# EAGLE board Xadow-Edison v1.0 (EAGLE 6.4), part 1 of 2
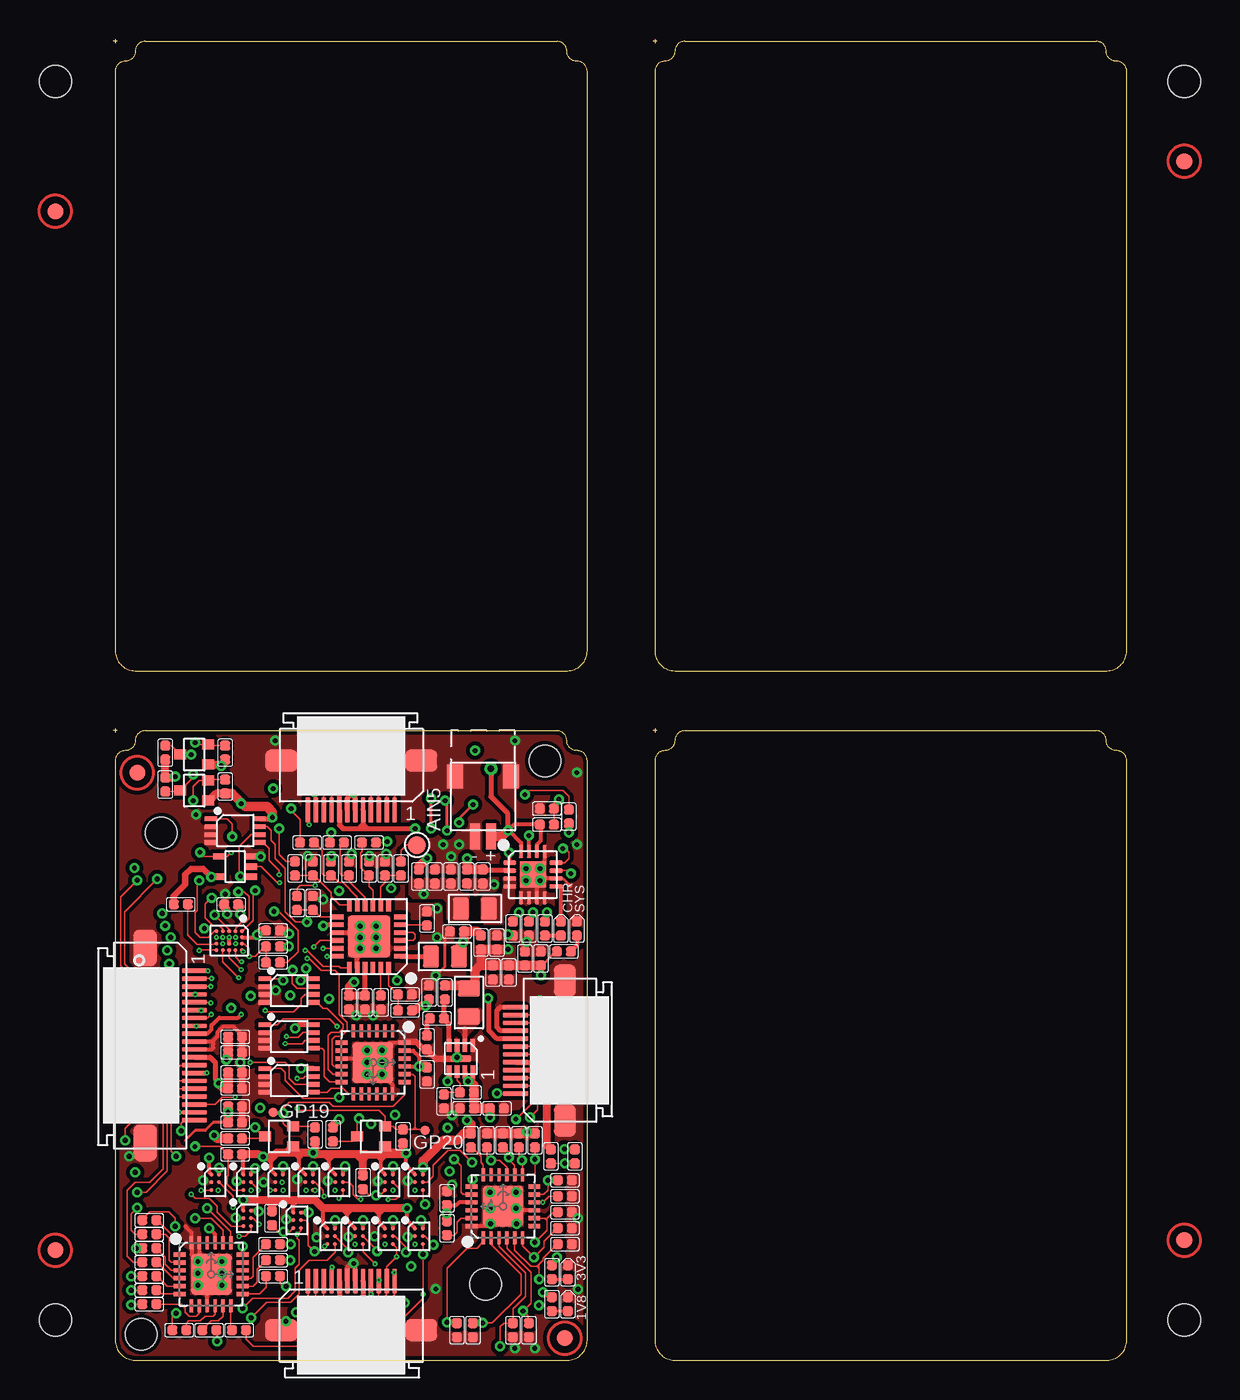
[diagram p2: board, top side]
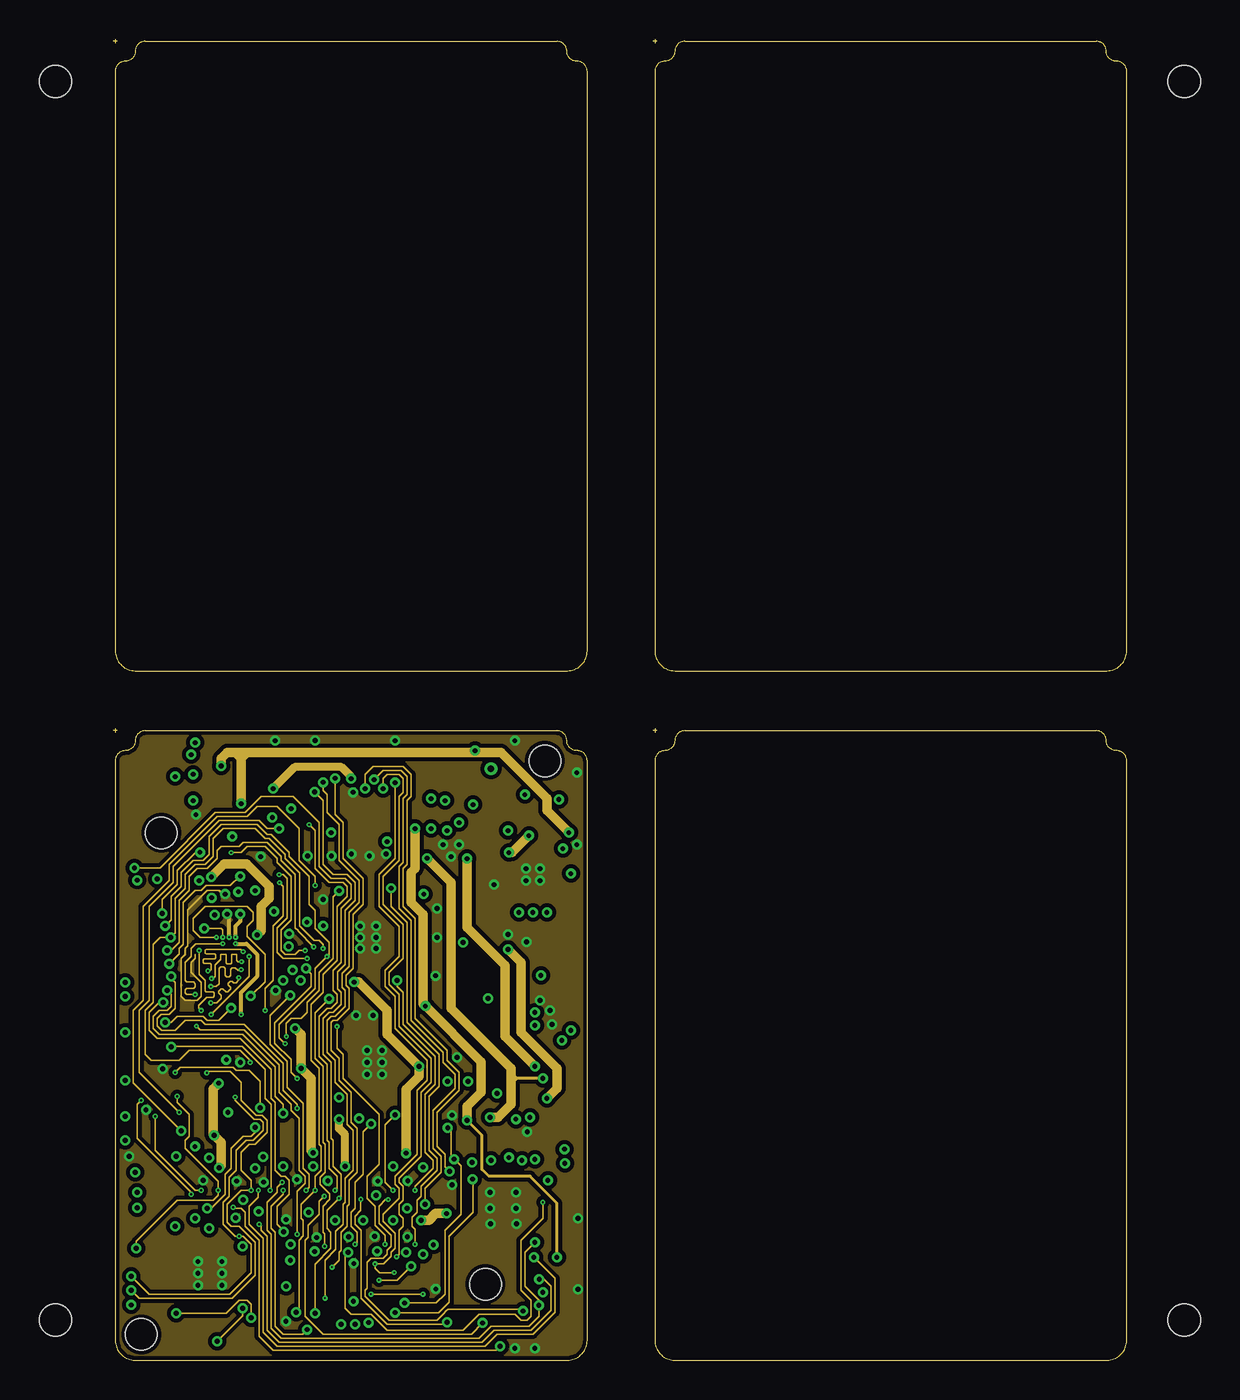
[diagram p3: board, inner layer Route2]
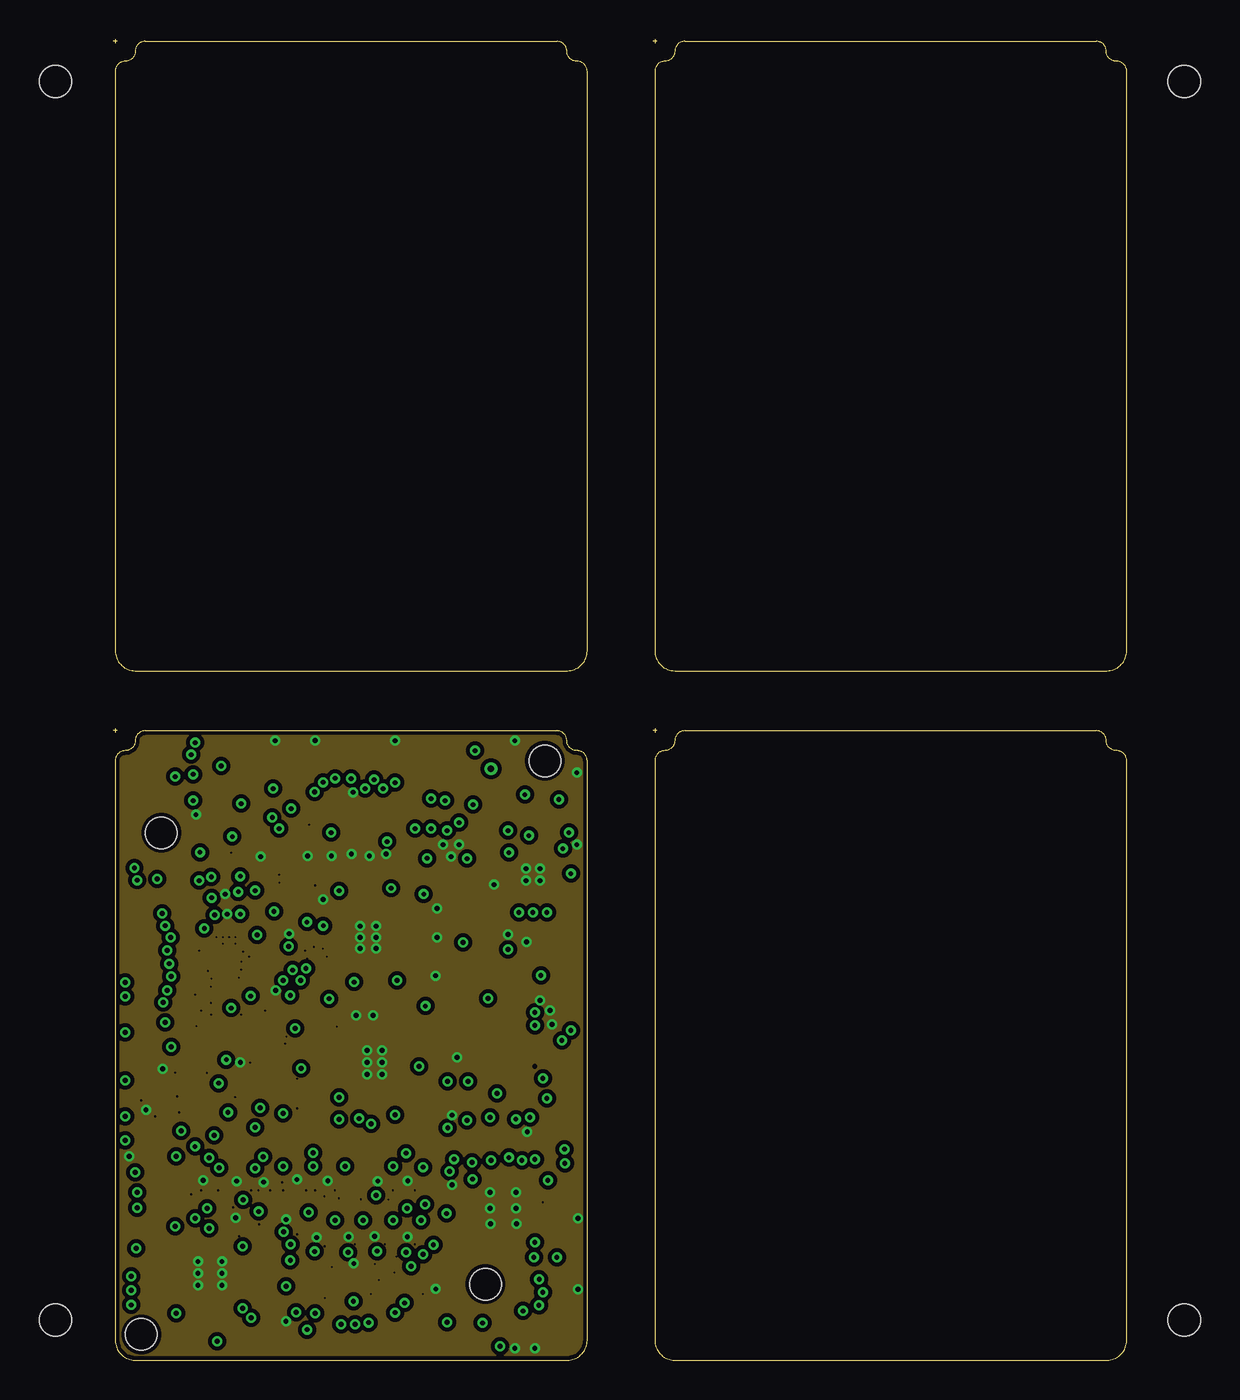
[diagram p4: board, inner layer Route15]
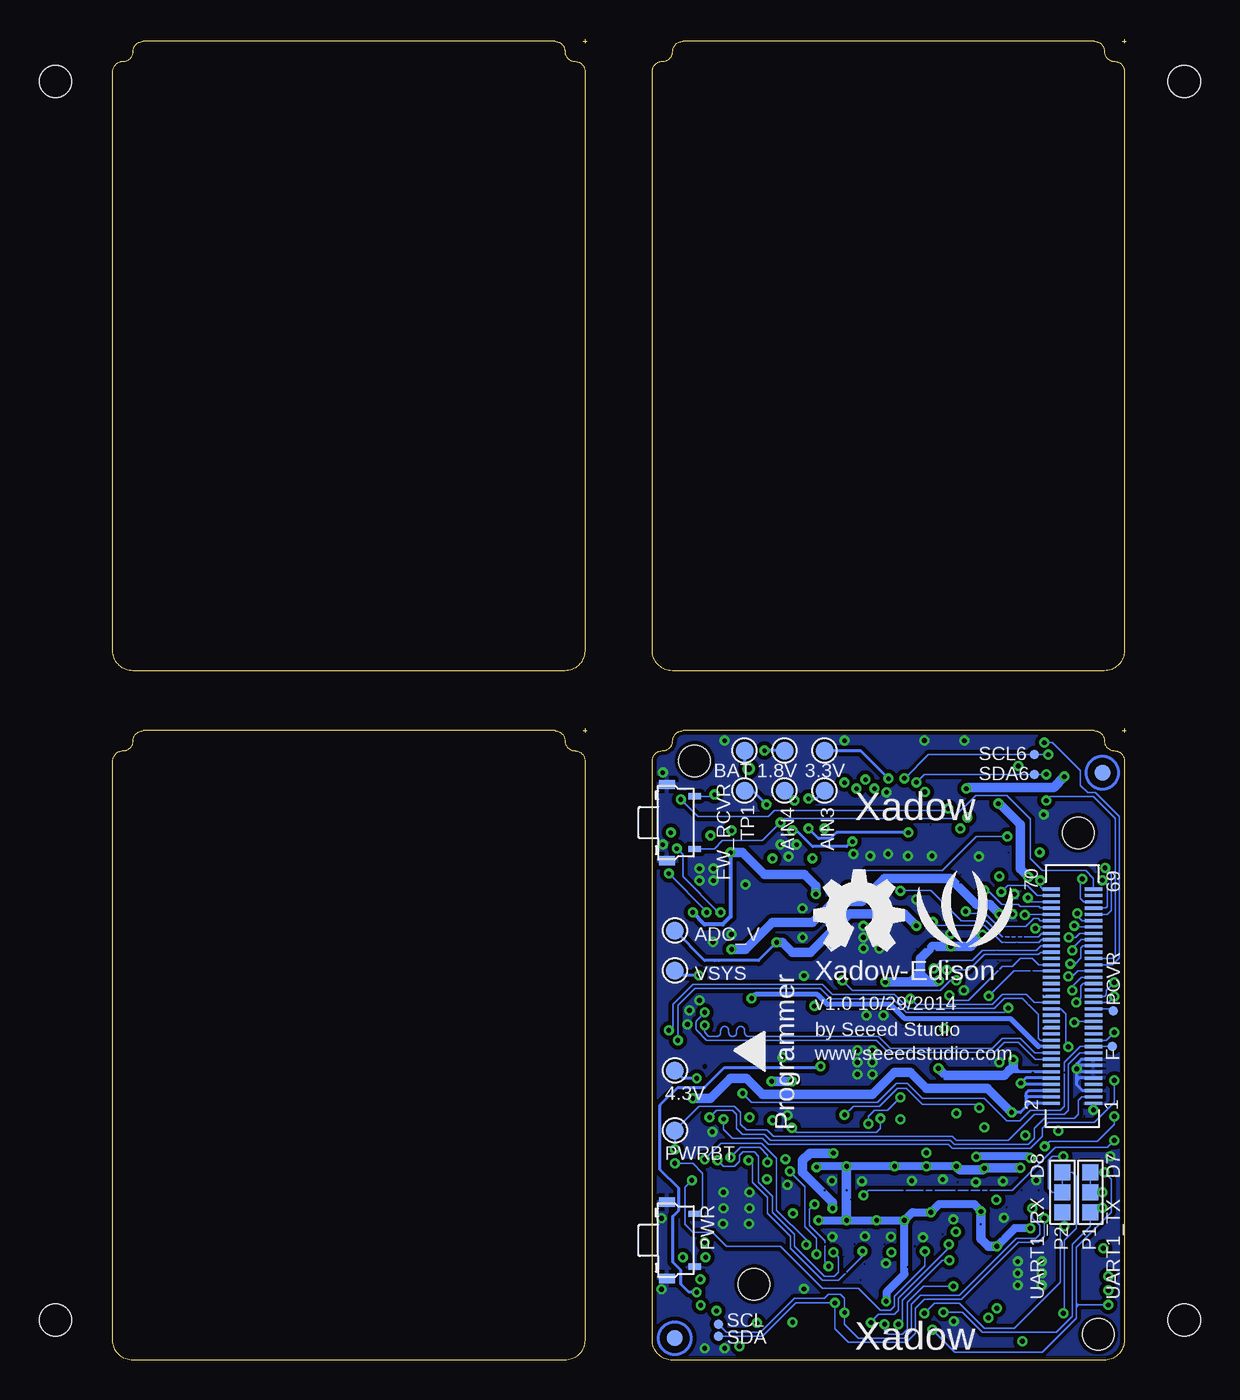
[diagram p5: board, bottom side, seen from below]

Size 64.42 x 83.95 mm. Coordinates in mm from the lower left corner, seen from the top.
Outline: 69 segments
Copper layers [2:(1+(2*15)+16):15]: Top 0.035mm / dielectric 0.2mm / Route2 0.0175mm / dielectric 0.3mm / Route15 0.0175mm / dielectric 0.2mm / Bottom 0.035mm
Design rules "SeeedStudio_4layer_DRU_no_angle_20140221 *": minimum track width 4mil, minimum drill 4mil, track to track 6mil, track to pad 6mil, pad to pad 6mil, via to via 6mil, smd to smd 0mil, copper to edge 10mil, drill to drill 10mil, minimum pad ring 6mil, minimum via ring 4mil, stop-mask expansion 2mil, vias tented up to drill 25mil, thermal gap 10mil
Holes 2 mm at 3.06,33.52 23.66,4.83 27.44,38.09 1.79,1.64
Holes 2.03 mm at -3.68,81.28 -3.68,2.54 68.07,81.28 68.07,2.54
tKeepout: area 21.8,2.9 to 25.6,6.7; area 1.2,31.6 to 5,35.4
bKeepout: area 1.2,31.6 to 5,35.4
tRestrict: area 22.9,28.1 to 23,29.2; area 22,22.7 to 23.2,22.8; area 21,25.1 to 21.1,26.2

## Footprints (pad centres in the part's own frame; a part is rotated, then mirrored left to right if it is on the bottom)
TP-D45MIL = smd 1.143 x 1.143: T 0,0
LED-0402 = smd 0.635 x 0.635: + -0.445,0; - 0.445,0
C0402 = smd 0.635 x 0.635: 1 -0.445,0; 2 0.445,0
TP-D23MIL = smd 0.6 x 0.6: T 0,0
4P-SMD-L4.5*W3.8*H1.8MM-90D = smd 0.4 x 0.8: 1 -1.675,-1.277; 2 1.675,-1.277 | smd 0.6 x 1: S1 -2.425,0.5; S2 2.425,0.5
70PIN-SMD-L16.64*W3.38*H3.12MM = smd 0.2 x 1.1: 1 -6.8,-1.34; 2 -6.8,1.34; 3 -6.4,-1.34; 4 -6.4,1.34; 5 -6,-1.34; 6 -6,1.34; 7 -5.6,-1.34; 8 -5.6,1.34; 9 -5.2,-1.34; 10 -5.2,1.34; 11 -4.8,-1.34; 12 -4.8,1.34; 13 -4.4,-1.34; 14 -4.4,1.34; 15 -4,-1.34; 16 -4,1.34; 17 -3.6,-1.34; 18 -3.6,1.34; 19 -3.2,-1.34; 20 -3.2,1.34; 21 -2.8,-1.34; 22 -2.8,1.34; 23 -2.4,-1.34; 24 -2.4,1.34; 25 -2,-1.34; 26 -2,1.34; 27 -1.6,-1.34; 28 -1.6,1.34; 29 -1.2,-1.34; 30 -1.2,1.34; 31 -0.8,-1.34; 32 -0.8,1.34; 33 -0.4,-1.34; 34 -0.4,1.34; 35 0,-1.34; 36 0,1.34; 37 0.4,-1.34; 38 0.4,1.34; 39 0.8,-1.34; 40 0.8,1.34; 41 1.2,-1.34; 42 1.2,1.34; 43 1.6,-1.34; 44 1.6,1.34; 45 2,-1.34; 46 2,1.34; 47 2.4,-1.34; 48 2.4,1.34; 49 2.8,-1.34; 50 2.8,1.34; 51 3.2,-1.34; 52 3.2,1.34; 53 3.6,-1.34; 54 3.6,1.34; 55 4,-1.34; 56 4,1.34; 57 4.4,-1.34; 58 4.4,1.34; 59 4.8,-1.34; 60 4.8,1.34; 61 5.2,-1.34; 62 5.2,1.34; 63 5.6,-1.34; 64 5.6,1.34; 65 6,-1.34; 66 6,1.34; 67 6.4,-1.34; 68 6.4,1.34; 69 6.8,-1.34; 70 6.8,1.34
20P-0.5 = smd 0.3 x 1.6: 1 -4.75,3.127; 2 -4.25,3.127; 3 -3.75,3.127; 4 -3.25,3.127; 5 -2.75,3.127; 6 -2.25,3.127; 7 -1.75,3.127; 8 -1.25,3.127; 9 -0.75,3.127; 10 -0.25,3.127; 11 0.25,3.127; 12 0.75,3.127; 13 1.25,3.127; 14 1.75,3.127; 15 2.25,3.127; 16 2.75,3.127; 17 3.25,3.127; 18 3.75,3.127; 19 4.25,3.127; 20 4.75,3.127 | smd 2.3 x 1.5: P1 -6.2,0; P2 6.2,0
12P-0.5-NEW = smd 0.3 x 1.6: 1 -2.75,3.127; 2 -2.25,3.127; 3 -1.75,3.127; 4 -1.25,3.127; 5 -0.75,3.127; 6 -0.25,3.127; 7 0.25,3.127; 8 0.75,3.127; 9 1.25,3.127; 10 1.75,3.127; 11 2.25,3.127; 12 2.75,3.127 | smd 2.032 x 1.397: P1 -4.445,0; P2 4.445,0
2P-SMD-1.0-90D = smd 1.524 x 1.016: 3 -3.429,1.778; 4 -3.429,-1.778 | smd 1.651 x 0.635: + 0.381,0.508; - 0.381,-0.508
L0805 = smd 1.016 x 1.397: 1 -0.889,0; 2 0.889,0
3P-SMD-4.1X1.5 = smd 1.016 x 1.016: 00 -1.27,0; 11 1.27,0; MM 0,0
ROUND-MARK-1.0 = smd 1.016 x 1.016: P$1 0,0
SOT-323 = smd 0.635 x 0.762: 1 -0.635,-0.889; 2 0.635,-0.889; 3 0,0.889
R0402 = smd 0.635 x 0.635: 1 -0.445,0; 2 0.445,0
S-PVQFN-N24 = smd 0.8 x 0.3: 1 -2,1.25; 2 -2,0.75; 3 -2,0.25; 4 -2,-0.25; 5 -2,-0.75; 6 -2,-1.25; 13 2,-1.25; 14 2,-0.75; 15 2,-0.25; 16 2,0.25; 17 2,0.75; 18 2,1.25 | smd 0.3 x 0.8: 7 -1.25,-2; 8 -0.75,-2; 9 -0.25,-2; 10 0.25,-2; 11 0.75,-2; 12 1.25,-2; 19 1.25,2; 20 0.75,2; 21 0.25,2; 22 -0.25,2; 23 -0.75,2; 24 -1.25,2 | smd 2.7 x 2.7: P$25 0,0
R-XBGA-N6 = smd 0.25 x 0.25: 1 -0.25,0.5; 2 -0.25,0; 3 -0.25,-0.5; 4 0.25,-0.5; 5 0.25,0; 6 0.25,0.5
QFN24 = smd 0.8 x 0.26: 1 -2,1.25; 2 -2,0.75; 3 -2,0.25; 4 -2,-0.25; 5 -2,-0.75; 6 -2,-1.25; 13 2,-1.25; 14 2,-0.75; 15 2,-0.25; 16 2,0.25; 17 2,0.75; 18 2,1.25 | smd 0.26 x 0.8: 7 -1.25,-2; 8 -0.75,-2; 9 -0.25,-2; 10 0.25,-2; 11 0.75,-2; 12 1.25,-2; 19 1.25,2; 20 0.75,2; 21 0.25,2; 22 -0.25,2; 23 -0.75,2; 24 -1.25,2 | smd 2.6 x 2.6: E 0.02,-0.01
R-XBGA-N20 = smd 0.25 x 0.25: 1 -0.6,0.8; 2 -0.2,0.8; 3 0.2,0.8; 4 0.6,0.8; 5 -0.6,0.4; 6 -0.2,0.4; 7 0.2,0.4; 8 0.6,0.4; 9 -0.6,0; 10 -0.2,0; 11 0.2,0; 12 0.6,0; 13 -0.6,-0.4; 14 -0.2,-0.4; 15 0.2,-0.4; 16 0.6,-0.4; 17 -0.6,-0.8; 18 -0.2,-0.8; 19 0.2,-0.8; 20 0.6,-0.8
US-8 = smd 0.3 x 0.8: 1 -0.75,-1.55; 2 -0.25,-1.55; 3 0.25,-1.55; 4 0.75,-1.55; 5 0.75,1.55; 6 0.25,1.55; 7 -0.25,1.55; 8 -0.75,1.55
SOT-353 = smd 0.4 x 0.8: 1 -0.65,-1; 2 0,-1; 3 0.65,-1; 4 0.65,1; 5 -0.65,1
QFN16 = smd 0.85 x 0.28: 1 -1.475,0.75; 2 -1.475,0.25; 3 -1.475,-0.25; 4 -1.475,-0.75; 9 1.475,-0.75; 10 1.475,-0.25; 11 1.475,0.25; 12 1.475,0.75 | smd 0.28 x 0.85: 5 -0.75,-1.475; 6 -0.25,-1.475; 7 0.25,-1.475; 8 0.75,-1.475; 13 0.75,1.475; 14 0.25,1.475; 15 -0.25,1.475; 16 -0.75,1.475 | smd 1.65 x 1.65: PAD 0,0
DFN-8L = smd 0.8 x 0.3: 1 -0.827,0.75; 2 -0.827,0.25; 3 -0.827,-0.25; 4 -0.827,-0.75; 5 0.827,-0.75; 6 0.827,-0.25; 7 0.827,0.25; 8 0.827,0.75 | smd 0.45 x 1.3: 9 0,0

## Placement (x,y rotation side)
1.8V  [TP-D45MIL]  21.72,38.73 0 bottom
1V8  red  [LED-0402]  28.89,3.56 90 top
3.3V  [TP-D45MIL]  19.18,38.73 0 bottom
3V3  blue  [LED-0402]  28.89,5.59 90 top
4.3V  [TP-D45MIL]  28.7,18.41 0 bottom
ADC_V  [TP-D45MIL]  28.7,27.3 0 bottom
AIN3  [TP-D45MIL]  19.18,36.2 0 bottom
AIN4  [TP-D45MIL]  21.72,36.2 0 bottom
AIN5  [TP-D45MIL]  19.3,32.74 0 top
BAT  [TP-D45MIL]  24.26,38.73 0 bottom
C3  10uF  [C0402]  14.99,22.73 270 top
C4  100nF  [C0402]  16,22.73 270 top
C5  10uF  [C0402]  21.84,27.24 180 top
C6  100nF  [C0402]  24.38,26.54 90 top
C7  10uF  [C0402]  20.07,23.37 90 top
C8  100pF  [C0402]  12.7,29.06 270 top
C9  100pF  [C0402]  12.7,31.24 270 top
C10  100pF  [C0402]  13.84,31.24 270 top
C11  100pF  [C0402]  14.99,31.24 270 top
C12  100pF  [C0402]  16.26,31.24 270 top
C13  100pF  [C0402]  17.27,31.24 270 top
C14  100nF  [C0402]  10.16,27.3 0 top
C15  100nF  [C0402]  7.49,28.96 180 top
C16  100nF  [C0402]  21.21,10.29 90 top
C17  100nF  [C0402]  19.94,18.16 270 top
C19  10uF  [C0402]  25.15,24.64 270 top
C20  10uF  [C0402]  24.13,24.64 270 top
C21  100nF  [C0402]  26.16,25.53 90 top
C22  100nF  [C0402]  27.18,25.53 90 top
C23  10uF  [C0402]  22.48,16 180 top
C24  10uF  [C0402]  24.38,16 0 top
C25  10uF  [C0402]  22.48,30.73 90 top
C26  10uF  [C0402]  23.49,30.73 90 top
C27  10uF  [C0402]  21.46,30.73 90 top
C28  10uF  [C0402]  20.45,30.73 90 top
C29  10uF  [C0402]  7.75,15.11 0 top
C30  10uF  [C0402]  7.75,16.13 0 top
C31  10uF  [C0402]  7.75,17.27 0 top
C32  10uF  [C0402]  7.75,18.29 0 top
C33  10uF  [C0402]  7.75,19.56 0 top
C34  10uF  [C0402]  7.75,20.55 0 top
CHR  green  [LED-0402]  28.45,27.43 90 top
F  [TP-D23MIL]  0.89,19.94 0 bottom
FW_RCVR  311020035  [4P-SMD-L4.5*W3.8*H1.8MM-90D]  28.7,34.16 90 bottom
GP19  [TP-D23MIL]  10.16,15.75 0 top
GP20  [TP-D23MIL]  19.81,14.61 0 top
J1  DF40C(2.0)-70DS-0.4V(51)  [70PIN-SMD-L16.64*W3.38*H3.12MM]  3.43,23.13 90 bottom
J2  FH12-20S-0.5SH(55)  [20P-0.5]  2.03,20 270 top
J3  320060003／／FH12-12S-0.5SH(55)  [12P-0.5-NEW]  15.13,1.91 0 top
J4  320060003／／FH12-12S-0.5SH(55)  [12P-0.5-NEW]  15.13,38.1 180 top
J8  320110054  [2P-SMD-1.0-90D]  23.49,33.66 270 top
J9  320060003／／FH12-12S-0.5SH(55)  [12P-0.5-NEW]  28.7,19.68 90 top
L1  120R  [L0805]  21.08,25.65 180 top
L2  2.2uH  [L0805]  22.61,22.73 90 top
L3  2.2uH  [L0805]  22.99,28.7 180 top
P1  [3P-SMD-4.1X1.5]  2.29,10.67 90 bottom
P2  [3P-SMD-4.1X1.5]  4.06,10.67 90 bottom
P3  DNP  [ROUND-MARK-1.0]  28.7,1.4 0 bottom
P4  [ROUND-MARK-1.0]  not placed on the board
P5  [ROUND-MARK-1.0]  not placed on the board
P6  [ROUND-MARK-1.0]  not placed on the board
P7  [ROUND-MARK-1.0]  not placed on the board
P11  DNP  [ROUND-MARK-1.0]  28.7,1.4 0 top
P12  √  [ROUND-MARK-1.0]  1.52,37.34 0 bottom
P13  √  [ROUND-MARK-1.0]  1.52,37.34 0 top
PCVR  [TP-D23MIL]  0.83,22.19 0 bottom
PWR  311020035  [4P-SMD-L4.5*W3.8*H1.8MM-90D]  28.7,7.62 90 bottom
PWRBT  [TP-D45MIL]  28.7,14.61 0 bottom
Q1  BSS138LT3G  [SOT-323]  16.38,14.22 90 top
Q2  BSS138LT3G  [SOT-323]  10.54,14.22 90 top
Q3  BSS138LT3G  [SOT-323]  5.14,36.2 90 top
Q4  BSS138LT3G  [SOT-323]  5.14,38.48 90 top
R1  47K_1%  [R0402]  20.57,21.72 180 top
R2  1.8K  [R0402]  7.11,36.45 270 top
R3  3.3K  [R0402]  3.3,36.58 90 top
R4  0R  [R0402]  19.94,28.07 90 top
R5  0R  [R0402]  17.02,22.73 270 top
R6  22K_1%  [R0402]  18.54,23.24 0 top
R7  22K_1%  [R0402]  18.54,22.23 0 top
R8  33R  [R0402]  11.68,29.06 90 top
R9  33R  [R0402]  11.56,31.24 90 top
R10  33R  [R0402]  12.32,32.89 180 top
R11  33R  [R0402]  14.22,32.89 180 top
R12  33R  [R0402]  16.26,32.89 0 top
R13  33R  [R0402]  18.29,31.24 90 top
R14  10K  [R0402]  4.29,28.97 180 top
R15  10K  [R0402]  10.16,26.29 180 top
R16  10K  [R0402]  21.84,1.91 90 top
R17  10K  [R0402]  22.86,1.91 90 top
R18  10K  [R0402]  28.7,10.41 0 top
R19  10K  [R0402]  26.8,13.97 90 top
R20  10K  [R0402]  25.78,13.97 90 top
R21  10K  [R0402]  24.77,13.97 90 top
R22  10K  [R0402]  23.75,13.97 90 top
R23  0R  [R0402]  10.16,25.27 0 top
R24  10K  [R0402]  22.48,17.02 180 top
R25  NC  [R0402]  21.02,16.45 270 top
R26  510K  [R0402]  21.08,23.37 270 top
R27  47K_1%  [R0402]  19.94,20.19 270 top
R28  5.1K  [R0402]  25.4,27.43 270 top
R29  5.1K  [R0402]  26.42,27.43 270 top
R30  47K  [R0402]  10.08,9.02 90 top
R31  470  [R0402]  27.43,27.43 270 top
R32  10K  [R0402]  27.81,12.95 270 top
R33  0R  [R0402]  19.43,30.73 270 top
R34  100R  [R0402]  29.34,12.95 90 top
R35  100R  [R0402]  28.96,34.54 270 top
R36  1.8K  [R0402]  7.11,38.61 270 top
R37  0R  [R0402]  23.37,26.54 90 top
R38  1.8K  [R0402]  27.88,5.59 270 top
R39  510R  [R0402]  27.88,3.56 270 top
R40  1.8K  [R0402]  18.41,14.22 270 top
R41  3.3K  [R0402]  13.97,14.35 90 top
R42  1.8K  [R0402]  12.83,14.35 270 top
R43  3.3K  [R0402]  7.75,14.1 180 top
R44  10K  [R0402]  21.21,8.38 90 top
R45  10K  [R0402]  22.73,13.97 90 top
R46  47K  [R0402]  15.88,11.3 90 top
R47  47K  [R0402]  7.75,13.08 0 top
R48  10K  [R0402]  28.7,7.37 180 top
R49  10K  [R0402]  28.7,9.4 180 top
R50  10K  [R0402]  28.7,8.38 180 top
R51  10K  [R0402]  26.42,1.91 90 top
R52  10K  [R0402]  28.7,11.43 0 top
R53  10K  [R0402]  25.4,1.91 90 top
R54  47K  [R0402]  10.16,7.37 0 top
R55  47K  [R0402]  10.16,6.35 0 top
R56  47K  [R0402]  10.16,5.33 0 top
R57  47K  [R0402]  8,1.91 0 top
R58  47K  [R0402]  4.19,1.91 180 top
R59  47K  [R0402]  2.29,8.89 0 top
R60  47K  [R0402]  2.29,8 0 top
R61  47K  [R0402]  2.29,3.56 0 top
R62  47K  [R0402]  2.29,5.33 0 top
R63  47K  [R0402]  2.29,7.11 0 top
R64  47K  [R0402]  6.1,1.91 0 top
R65  47K  [R0402]  2.29,6.22 0 top
R66  47K  [R0402]  2.29,4.45 0 top
R67  3.3K  [R0402]  3.3,38.61 270 top
R68  1M_1%  [R0402]  27.56,34.04 0 top
R69  1M_1%  [R0402]  27.56,35.05 180 top
R70  3.3K  [R0402]  28.64,25.97 0 top
SCL  [TP-D23MIL]  25.91,2.29 0 bottom
SCL6  [TP-D23MIL]  5.84,38.48 0 bottom
SDA  [TP-D23MIL]  25.91,1.52 0 bottom
SDA6  [TP-D23MIL]  5.84,37.21 0 bottom
SYS  White  [LED-0402]  29.46,27.43 90 top
TP1  [TP-D45MIL]  24.26,36.2 0 bottom
U2  ADS7951SBRGE  [S-PVQFN-N24]  16.26,26.92 180 top
U3  SN74LVC1T45YZPR  [R-XBGA-N6]  17.53,7.87 0 top
U4  PCAL9555AHF  [QFN24]  24.77,9.78 90 top
U5  SN74LVC1T45YZPR  [R-XBGA-N6]  19.43,11.3 0 top
U6  SN74LVC1T45YZPR  [R-XBGA-N6]  19.43,7.87 0 top
U7  SN74LVC1T45YZPR  [R-XBGA-N6]  11.68,8.89 0 top
U8  SN74LVC1T45YZPR  [R-XBGA-N6]  12.45,11.3 0 top
U9  SN74LVC1T45YZPR  [R-XBGA-N6]  14.35,11.3 0 top
U10  TXS0206-29YFPRB  [R-XBGA-N20]  7.37,26.67 270 top
U11  SN74LVC1T45YZPR  [R-XBGA-N6]  15.62,7.87 0 top
U12  SN74LVC2G53  [US-8]  11.18,17.78 270 top
U13  SN74AUP1G125DCKR  [SOT-353]  7.75,31.37 90 top
U14  SN74LVC2G53  [US-8]  11.18,20.57 270 top
U15  SN74LVC2G53  [US-8]  11.18,23.5 270 top
U16  SN74LVC2G53  [US-8]  7.75,33.66 270 top
U17  PCAL9555AHF  [QFN24]  16.51,18.92 270 top
U18  PCAL9535AHF  [QFN24]  6.22,5.46 0 top
U19  ETA6003Q3Q  [QFN16]  26.67,30.86 0 top
U22  SN74LVC1T45YZPR  [R-XBGA-N6]  17.53,11.3 0 top
U23  SN74LVC1T45YZPR  [R-XBGA-N6]  8.51,11.3 0 top
U24  SN74LVC1T45YZPR  [R-XBGA-N6]  10.54,11.3 0 top
U25  SN74LVC1T45YZPR  [R-XBGA-N6]  13.84,7.87 0 top
U26  SN74LVC1T45YZPR  [R-XBGA-N6]  6.48,11.3 0 top
U27  SN74LVC1T45YZPR  [R-XBGA-N6]  8.51,9.02 0 top
U28  ETA3410D2I-T  [DFN-8L]  22.1,19.18 270 top
U$13  [OSHW_FILLX200_NOTEXT]  19.81,26.04 0 bottom
U$14  [LOGO_SILK]  10.29,27.94 0 bottom
VSYS  [TP-D45MIL]  28.7,24.77 0 bottom

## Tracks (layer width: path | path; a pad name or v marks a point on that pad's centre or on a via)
ADC_VCC  (via drill 0.3 pad 0.64)
  Top 0.305: U2.14 13.41,27.67 v13.35,27.61
  Top 0.508: L1.1 21.97,26.29 v22.22,26.54
  Top 0.61: v22.22,26.54 22.29,26.61 C5.1 23.11,27.24 R37.2
  Bottom 0.203: v22.22,26.54 23.37,25.4 25.91,25.4 26.16,25.4 26.8,25.4 ADC_V.T
  Bottom 0.61: v22.22,26.54 21.84,26.54 21.21,25.91 20.07,25.91 17.6,28.37 14.11,28.37 v13.35,27.61
AIN0  (via drill 0.1 pad 0.25 layers 1-2, 0.3 pad 0.64)
  Top 0.102: R8.2 11.68,29.97 11.89,30.18 v12.83,30.18 | 4.57,15.24 4.52,15.24 4.32,15.04 v4.32,14.58
  Top 0.203: 4.57,15.24 J2.20
  Route2 0.102: v12.83,30.18 12.83,30.73 11.81,31.75 11.81,33.78 10.41,35.19 9.15,35.19 8.51,34.54 6.6,34.54 3.56,31.5 3.56,30.48 1.91,28.83 1.91,22.86 1.27,22.23 1.27,17.63 v4.32,14.58
AIN1  (via drill 0.1 pad 0.25 layers 1-2, 0.3 pad 0.64)
  Top 0.102: J2.19 v4.19,15.75 | R9.2 10.99,31.69 10.54,32.13 v10.54,33.78
  Route2 0.102: v10.54,33.78 9.78,33.78 9.27,34.29 6.73,34.29 3.81,31.37 3.81,30.35 2.29,28.83 2.29,22.86 1.65,22.23 1.65,18.29 v4.19,15.75
AIN2/BAT  (via drill 0.3 pad 0.64)
  Top 0.102: R68.2 R69.1 28,35.5 28.14,35.64 v28.32,35.64 | R10.2 11.88,34.35 11.3,34.92 v11.3,35.05
  Bottom 0.102: v11.3,35.05 11.43,34.92 22.35,34.92 22.73,34.54 27.23,34.54 v28.32,35.64
  pour Top (isolate 0.254, no thermals): 24.13,33.53 23.88,33.66 24,33.53
AIN3  (via drill 0.3 pad 0.64)
  Top 0.102: R11.2 13.78,33.47 v13.84,33.53
  Top 0.203: v20.19,33.78 v20.19,35.69
  Bottom 0.203: v13.84,33.53 18.41,33.53 18.8,33.15 19.56,33.15 v20.19,33.78 | v20.19,35.69 19.68,35.69 AIN3.T
AIN4  (via drill 0.3 pad 0.64)
  Top 0.102: R12.2 17.34,32.89 v17.4,32.96
  Top 0.203: v21.21,33.66 21.21,35.43 v21.08,35.56
  Bottom 0.203: AIN4.T v21.08,35.56 | v17.4,32.96 17.46,32.96 17.78,32.64 19.94,32.64 20.95,33.66 v21.21,33.66
AIN5
  Top 0.102: R13.2 18.29,32.38 18.64,32.74 AIN5.T
BAT  (via drill 0.3 pad 0.64, 0.41 pad 0.81)
  Top 0.203: 24.95,34.86 25.02,34.8
  Top 0.254: U19.14 26.92,32.76 27.18,33.02 27.18,33.97 R68.1 25.46,34.04 25.11,33.69 25.92,32.88 U19.16
  Top 0.305: v24,37.59 24,35.81 24.95,34.86 25.08,34.73 v25.08,33.66
  Top 0.61: J8.+ 24.7,33.27 v25.08,33.66 25.11,33.69
  Bottom 0.203: BAT.T 24.26,37.85 v24,37.59
CLKB  (via drill 0.1 pad 0.25 layers 1-2)
  Top 0.102: J2.4 v5.2,23.25 v5.21,23.24 | U10.15 v6.96,26.47
  Route2 0.102: v6.96,26.47 5.24,26.47 4.95,26.18 4.95,25.65 4.57,25.27 4.57,24.13 4.67,24.03 5.1,24.03 5.21,23.93 5.21,23.73 5.1,23.62 4.67,23.62 4.57,23.52 4.57,23.34 4.67,23.24 v5.21,23.24
CMDB  (via drill 0.1 pad 0.25 layers 1-2)
  Top 0.102: J2.3 v6.2,23.75 | U10.12 7.37,25.58 v8.13,24.82
  Route2 0.102: v6.2,23.75 6.55,23.75 6.73,23.93 6.73,24.9 6.82,24.98 7.02,24.98 7.11,24.9 7.11,24.46 7.2,24.37 7.38,24.37 7.47,24.46 7.47,24.84 7.57,24.94 7.75,24.94 7.92,24.77 8.08,24.77 v8.13,24.82
D7  (via drill 0.1 pad 0.25 layers 1-2, 0.3 pad 0.64)
  Top 0.102: U24.4 v10.79,10.79 | R61.1 1.19,3.56 v1.14,3.5
  Route2 0.102: v10.79,10.79 10.79,10.54 10.03,9.78 10.03,8.38 10.29,8.13 10.29,2.16 10.79,1.65 12.03,1.65 v12.32,1.94
  Bottom 0.102: 2.29,10.67 P1.11 v1.4,11.94 0.95,11.49 0.95,9.4 3.17,7.18 3.17,3.62 | v12.32,1.94 10.88,0.51 5.33,0.51 3.17,2.67 3.17,3.37 | v1.14,3.5 3.04,3.5 | 3.06,3.5 3.16,3.5 3.17,3.49 | 3.17,3.37 3.17,3.49 | 3.17,3.49 3.17,3.62 | 3.04,3.5 3.06,3.5 | 3.06,3.5 3.17,3.62 | 3.04,3.5 3.17,3.37
D8  (via drill 0.3 pad 0.64)
  Top 0.102: U25.4 14.09,6.85 13.59,6.35 12.45,6.35 11.81,5.71 11.81,4.22 11.27,3.68 9.75,3.68 v8.76,2.69 | R58.2 3.75,2.73 v4,2.98
  Route2 0.102: v8.76,2.69 8.76,3.56 8.51,3.81 8,3.81 7.17,2.98 v4,2.98
  Bottom 0.102: 4.06,10.67 P2.11 3.43,11.94 3.17,11.68 3.17,8.38 3.94,7.62 3.94,3.05 v4,2.98
DAT0B  (via drill 0.1 pad 0.25 layers 1-2)
  Top 0.102: U10.16 6.97,25.32 v7.98,24.31 | J2.5 6.15,22.75 v6.2,22.71
  Route2 0.102: v7.98,24.31 7.98,24.16 7.8,23.98 7.64,23.98 7.54,24.08 7.44,24.08 7.31,23.95 7.31,23.85 7.47,23.7 7.47,23.59 7.27,23.39 7.16,23.39 6.96,23.6 6.85,23.6 6.71,23.45 6.71,23.34 6.86,23.19 6.86,22.99 6.58,22.71 v6.2,22.71
DAT1B  (via drill 0.1 pad 0.25 layers 1-2)
  Top 0.102: J2.6 5.56,22.25 v5.59,22.23 | U10.20 5.5,26.07 v5.46,26.04
  Route2 0.102: v5.46,26.04 5.46,24.51 5.84,24.13 5.84,23.47 5.92,23.39 6.35,23.39 6.41,23.33 6.41,23.14 6.33,23.06 5.94,23.06 5.43,22.55 5.43,22.39 v5.59,22.23
DAT2B  (via drill 0.1 pad 0.25 layers 1-2)
  Top 0.102: U10.4 8.17,26.05 v8.26,25.96 | J2.1 v6.01,24.75 v6.02,24.74
  Route2 0.102: 8.15,26.06 v8.26,25.96 8.1,26.11 5.89,26.11 5.84,26.06 5.84,25.86 5.89,25.81 6.45,25.81 6.5,25.76 6.5,25.55 6.45,25.5 5.77,25.5 5.71,25.45 5.71,25.27 5.77,25.22 6.15,25.22 6.22,25.15 6.22,24.83 6.13,24.74 v6.02,24.74
DAT3B  (via drill 0.1 pad 0.25 layers 1-2)
  Top 0.102: U10.8 7.77,25.64 8.08,25.32 v8.15,25.32 | J2.2 v6.24,24.25 v6.25,24.26
  Route2 0.102: v8.15,25.32 7.92,25.32 7.85,25.4 7.85,25.76 7.8,25.8 7.57,25.8 7.52,25.76 7.52,25.25 7.47,25.2 7.24,25.2 7.19,25.25 7.19,25.76 7.15,25.79 6.87,25.79 6.83,25.76 6.83,25.48 6.48,25.12 6.48,24.38 6.35,24.26 v6.25,24.26
EN_SPI_CLK
  Top 0.102: U12.5 13.6,17.03 13.84,17.27 14.61,17.27 14.67,17.21 14.7,17.18 14.95,16.92 U17.13
EN_SPI_FUN  (via drill 0.1 pad 0.25 layers 1-2)
  Top 0.102: U17.10 14.03,18.67 13.91,18.8 13.91,20.38 14.1,20.57 14.48,20.57 14.86,20.95 14.86,21.46 14.35,21.97 14.35,24.51 14.1,24.77 13.21,24.77 12.45,25.53 v12.32,25.53 | U16.5 9.54,32.91 9.91,32.54 9.91,31.75 10.54,31.11 v10.54,30.86
  Route2 0.102: v12.32,25.53 10.79,25.53 10.41,25.91 10.41,27.48 11.05,28.12 11.05,30.61 10.79,30.86 v10.54,30.86
EN_SPI_MISO
  Top 0.102: U17.11 13.96,18.17 13.65,18.48 13.65,20.64 13.84,20.83 14.35,20.83 14.61,21.08 14.61,21.34 13.59,22.35 13.34,22.35 12.94,22.75 U15.5
EN_SPI_MOSI
  Top 0.102: U17.12 13.76,17.67 13.4,18.03 13.4,19.68 13.3,19.78 13.27,19.81 13.26,19.82 U14.5
FAULT  (via drill 0.3 pad 0.64)
  Top 0.102: J9.1 24.4,16.93 v24.38,16.95
  Bottom 0.102: F.T 0.9,19.93 J1.19 2.93,19.93 3.94,18.92 3.94,16.13 4.19,15.88 6.1,15.88 6.77,15.2 7.58,15.2 9.02,16.64 12.95,16.64 13.91,17.59 14.61,17.59 15.81,16.38 18.29,16.38 23.81,16.38 v24.38,16.95
FW_RCVR  (via drill 0.3 pad 0.64)
  Top 0.203: v21.97,34.16 21.97,34.42 v22.86,35.31
  Bottom 0.102: 27.32,32.38 FW_RCVR.1 26.19,32.49 25.65,33.02 23.11,33.02 v21.97,34.16 21.72,34.42 11.05,34.42 9.58,35.89 7.6,35.89 6.1,34.38 6.1,31.88 5.33,31.11 2.59,31.11 2.09,30.61 J1.69
  Bottom 0.203: TP1.T 23.75,36.2 v22.86,35.31
GND  (via drill 0.1 pad 0.25 layers 1-2, 0.3 pad 0.64)
  Top 0.203: v20.57,26.87 21.03,26.87 21.08,26.92 | 21.08,26.92 C5.2 | C7.2 20.48,24.23 v20.48,24.43 v20.5,24.43 21.08,25.02 21.08,26.92 | U19.10 28.57,30.61 29.08,30.1
  Top 0.254: U19.13 27.42,31.54 v27.13,31.24 | U19.10 27.26,30.61 v27.13,30.48 26.92,30.27 U19.7 | U17.24 17.58,20.17 v17.09,19.68 | U17.9 15.89,19.17 v16.14,18.92 | U18.9 5.97,4.16 v5.38,4.75 | C11.1 14.99,32.03 v15.14,32.18 | U28.3 v21.85,19.26 v21.84,19.25 | v17.09,18.16 17.76,17.5 U17.18 | U18.23 5.47,6.36 v5.38,6.27 | 5.46,6.22 4.97,6.71 U18.24 4.97,8.11 4.57,8.51 | U4.9 25.73,9.53 v25.6,9.65 | U10.11 U10.10 | U4.24 23.84,8.53 v23.98,8.66 | J2.11 6.24,19.75 6.35,19.86 6.35,20.09 | 6.35,20.09 6.35,20.32 | 6.35,20.32 6.63,20.6 6.63,20.85 6.98,21.21 7.62,21.21 8.13,20.7 8.13,20.61 C34.2 | J2.10 6.28,20.25 6.35,20.32 | 6.35,20.09 6.2,20.24 | 28.51,23.94 J9.P2
  Top 0.305: C3.2 15.06,22.29 v15.44,21.91 | J4.6 15.38,35.96 v15.24,36.09 14.88,35.73 J4.7 | U2.20 15.51,25.97 v15.7,26.16 | J3.7 15.38,6.06 v15.29,6.15 15.16,6.15 14.88,5.86 J3.6 | U2.15 15.4,27.17 v15.7,26.87 | J9.9 24.63,20.93 24.38,21.18 24.38,22.23 24.59,22.43 J9.12
  Top 0.406: 19.93,19.75 20.52,19.15 21.74,19.15 v21.84,19.25 | R27.2 19.93,19.75 | 19.93,19.75 19.72,19.75 19.25,20.22 18.54,20.22 18.52,20.19 | C34.2 C33.2 C32.2 C31.2 | C30.2 C29.2
  Top 0.508: v26.24,30.48 26.29,30.48 U19.PAD | C15.2 7.05,28.77 7.24,28.57 v7.24,28.35 | C14.2 10.97,27.3 v11.18,27.1 | R19.2 26.4,14.41 v26.31,14.5
  Top 0.61: v23.95,9.65 24.63,9.65 U4.E | R22.2 R21.2 R20.2 26.23,14.41 v26.31,14.5
  Route2 0.102: v7.11,29.62 6.96,29.62 6.73,29.84 5.97,29.84 4.72,28.6 4.72,26.31 4.57,26.16 4.57,25.78 4.32,25.53 4.32,23.11 4.57,22.86 5.33,22.86 5.59,23.11 5.59,24 4.95,24.64 4.95,25.27 5.21,25.53 5.21,25.78
  Route2 0.254: U10.10 7.37,28.22 v7.24,28.35
  Bottom 0.203: J1.9 2.97,17.93 | 3,17.93 3.13,17.93 3.15,17.91 | J1.13 3.01,18.73 | 3.15,18.24 v3.15,18.52 3.15,18.59 | 3.15,18.59 3.01,18.73 | J1.11 3.06,18.33 | 3.06,18.33 3.15,18.24 | 3.06,18.33 3.06,18.35 3.12,18.41 | J1.15 2.87,19.13 3.15,18.85 3.15,18.59 | 3.01,18.73 3.01,18.76 3.05,18.8 | J1.1 v2.09,15.9 v2.08,15.9 | J1.5 2.78,17.13 3.15,17.5 3.15,17.75 | 3.15,17.75 3.15,17.91 | 3.15,17.91 3.15,18.09 | 3.15,18.09 3.15,18.24 | 2.97,17.93 3.15,17.75 | 2.97,17.93 3,17.93 | 3,17.93 3.15,18.09
  other vias: 5.71,11.43 7.84,11.38 13.64,11.4 16.81,11.38 18.72,11.4 9.56,11.32 11.67,11.48 7.77,9.04 10.99,8.94 12.93,7.8 14.96,7.85 16.61,7.87 18.69,7.85 25.63,8.66 23.95,10.67 25.6,10.67 6.91,6.27 6.91,5.51 6.91,4.75 5.38,5.51 16.52,21.91 16.14,19.68 16.14,18.16 17.09,18.92 15.7,27.58 16.71,26.16 16.71,26.87 16.71,27.58 26.24,31.24 26.26,26.58 20.59,28.7 24.21,30.23 25.1,27.05 25.53,39.37 12.34,32.05 13.87,32.05 16.28,32.05 21.54,15.57 29.54,9.02 10.97,2.46 1.02,12.95 10.29,39.37 26.8,0.76 25.53,0.76 12.83,39.38 17.91,39.37 17.34,32.17 13.34,29.29 10.33,23.5 7.37,26.87 5.26,34.67 9.37,32 21.54,11.15 29.46,32.77 29.46,37.34 21.46,32 20.5,4.52 29.54,4.51 21.97,32.77 20.95,32.77 8.08,18.92 27.76,22.23 27.13,22.86 27.89,21.34
  pour Top (isolate 0.254, rank 6, no thermals): -0.51,40.64 30.61,40.64 30.61,-0.64 -0.51,-0.64
  pour Bottom (isolate 0.254, rank 6): -0.51,40.64 30.61,40.64 30.61,-0.64 -0.51,-0.64
  pour Route2 (isolate 0.254, rank 6): -0.51,40.64 30.61,40.64 30.61,-0.64 -0.51,-0.64
  pour Route15 (isolate 0.254, rank 6): -0.51,40.64 30.61,40.64 30.61,-0.64 -0.51,-0.64
GP12  (via drill 0.3 pad 0.64)
  Top 0.102: 15.81,10.86 R46.1 16.26,10.48 v16.7,10.48 16.95,10.48 U22.3 | v0.76,24 1.14,24 1.78,23.37 1.78,17.02 1.4,16.64 1.4,15.37 0.76,14.73 v0.76,13.97
  Bottom 0.102: v16.7,10.48 16.38,10.79 7.24,10.79 4.51,13.53 1.21,13.53 v0.76,13.97 | J1.35 1.38,23.13 1.27,23.24 1.27,23.5 v0.76,24
GP13  (via drill 0.3 pad 0.64)
  Top 0.102: 7.37,13.14 R47.1 | U23.3 7.62,10.79 7.24,11.18 7.24,11.68 7.3,11.75 R47.1 | v0.76,23.11 1.02,23.11 1.4,22.73 1.4,17.53 0.76,16.89 v0.76,15.49 | v5.19,13.58 6.81,13.58 R47.1
  Bottom 0.102: J1.33 1.15,22.73 v0.76,23.11 | v0.76,15.49 0.76,14.99 1.85,13.89 4.88,13.89 v5.19,13.58
GP19  (via drill 0.3 pad 0.64)
  Top 0.102: U17.19 18.51,16.86 17.78,16.13 13.97,16.13 13.72,16.38 11.18,16.38 10.79,16 v10.79,15.68 10.79,15.06 11,14.86 Q2.2 12.76,14.86 R42.1
  Top 0.203: 10.1,15.68 GP19.T 10.22,15.68 v10.79,15.68
  Route2 0.102: v10.79,15.68 10.79,16.26 10.29,16.76 10.29,18.64 8.23,20.7 2.92,20.7 2.54,21.08 2.54,21.84 2.92,22.23 3.43,22.23 3.68,22.48 3.68,23.24 v3.43,23.5
  Bottom 0.102: J1.41 2.85,24.33 3.43,23.75 v3.43,23.5
GP20  (via drill 0.1 pad 0.25 layers 1-2, 0.3 pad 0.64)
  Top 0.102: R40.1 18.22,14.67 | R40.1 17.97,14.67 17.78,14.86 Q1.2 17.27,15.49 16.89,15.88 11.81,15.88 v11.68,16 | GP20.T 19.75,14.67 19.05,14.67 | U17.20 19.04,18.17 19.18,18.03 19.18,14.8 | 19.05,14.67 R40.1 | 19.18,14.8 19.05,14.67 | 19.18,14.78 19.18,14.73 | 19.18,14.8 19.18,14.78 | 19.18,14.78 19.28,14.68
  Route2 0.102: v11.68,16 11.68,16.26 10.79,17.14 10.79,18.86 8.32,21.34 5.84,21.34 5.59,21.59 4.57,21.59 3.94,20.95 3.08,20.95 2.79,21.25 2.79,21.72 3.05,21.97 3.56,21.97 3.94,22.35 3.94,24 3.68,24.26 v3.68,24.38
  Bottom 0.102: J1.43 3.08,24.73 3.43,24.38 v3.68,24.38
GP27/SCL6  (via drill 0.3 pad 0.64)
  Top 0.102: R36.1 6.1,39.05 Q4.2 5.33,39.12 v5.21,39.24
  Bottom 0.102: J1.45 0.91,25.13 0.46,25.58 0.46,34.54 1.98,36.07 2.46,36.07 2.92,36.53 2.92,37.47 4.7,39.24 v5.21,39.24
GP28/SDA6  (via drill 0.3 pad 0.64)
  Top 0.102: R2.1 6.1,36.89 Q3.2 5.46,36.83 5.08,36.45 v5.08,35.56
  Bottom 0.102: J1.47 0.89,25.53 0.71,25.7 0.71,34.42 2.11,35.81 4.83,35.81 v5.08,35.56
GP40  (via drill 0.1 pad 0.25 layers 1-2, 0.3 pad 0.64)
  Top 0.102: U12.7 12.19,18.03 12.07,17.91 v11.68,17.91
  Route2 0.102: v11.68,17.91 11.3,18.29 11.3,19.11 10.27,20.14 10.27,21.45 12.57,23.75 12.57,24.56 v12.24,24.89
  Bottom 0.102: J1.52 5.42,26.33 5.71,26.04 9.14,26.04 9.78,25.4 11.74,25.4 v12.24,24.89
GP41  (via drill 0.3 pad 0.64)
  Top 0.102: U16.7 9.78,33.91 10.03,33.66 10.03,33.02 10.29,32.77 10.29,31.88 10.92,31.24 10.92,28.5 11.58,27.84 v12.31,27.84
  Bottom 0.102: J1.54 5.38,26.73 5.56,26.54 7.92,26.54 9.02,27.64 12.1,27.64 v12.31,27.84
GP42  (via drill 0.3 pad 0.64)
  Top 0.102: U15.7 12.44,23.75 12.32,23.62 11.68,23.62 11.35,23.95 11.35,24.74 v11.41,24.79
  Bottom 0.102: J1.50 5.44,25.93 5.59,25.78 9.02,25.78 10.01,24.79 v11.41,24.79
GP43  (via drill 0.1 pad 0.25 layers 1-2, 0.3 pad 0.64)
  Top 0.102: U14.7 12.06,20.82 11.75,20.51 11.06,20.51 v11,20.57
  Route2 0.102: v14.36,29.83 13.97,29.44 13.97,25.53 13.08,24.64 13.08,23.5 12.32,22.73 12.32,22.1 11.94,21.72 11.3,21.72 11,21.41 v11,20.57
  Bottom 0.102: J1.56 5.36,27.13 5.59,26.9 7.87,26.9 8.89,27.91 10.49,27.91 12.42,29.84 14.35,29.84 v14.36,29.83
GP48  (via drill 0.1 pad 0.25 layers 1-2, 0.3 pad 0.64)
  Top 0.102: U24.3 v9.97,10.8 v9.97,10.79
  Route2 0.102: v3.68,19.91 3.71,19.94 8.19,19.94 9.65,18.48 9.65,16.64 10.03,16.26 10.03,10.86 v9.97,10.79
  Bottom 0.102: J1.32 4.17,22.33 3.86,22.02 3.86,20.09 v3.68,19.91
GP48CH  (via drill 0.1 pad 0.25 layers 1-2, 0.3 pad 0.64)
  Top 0.102: U24.5 v10.73,11.3 | U4.8 27.42,9.03 | 27.42,9.03 27.55,9.03 27.56,9.02 | 27.56,8.89 27.56,9.02 | R49.2 27.94,9.4 27.56,9.02 | 27.42,9.03 27.56,8.89 | 27.56,8.89 27.56,8.26 v26.8,7.49
  Route2 0.102: v10.73,11.3 10.41,10.99 10.41,10.67 9.78,10.03 9.78,8.26 10.03,8 10.03,2.03 10.67,1.4 23.24,1.4 24,2.16 26.42,2.16 27.05,2.79 v27.05,3.49 27.05,3.81 26.16,4.7 26.16,6.86 v26.8,7.49
GP49  (via drill 0.1 pad 0.25 layers 1-2, 0.3 pad 0.64)
  Top 0.102: U25.3 13.57,7.37 v13.44,7.24
  Route2 0.102: v13.72,22.97 12.83,22.09 12.83,19.18 13.34,18.67 13.34,13.84 13.46,13.72 13.46,11.94 13.15,11.62 13.15,11.19 13.77,10.57 13.77,10.21 13.34,9.78 13.34,8.13 13.44,8.03 v13.44,7.24
  Bottom 0.102: v13.72,22.97 13.35,22.61 8.51,22.61 7.87,23.24 6.35,23.24 5.84,22.73 J1.34
GP49CH  (via drill 0.1 pad 0.25 layers 1-2, 0.3 pad 0.64)
  Top 0.102: U25.5 14.94,7.04 v14.94,6.86 | R18.1 27.69,10.41 v27.3,10.03 U4.10
  Route2 0.102: v27.3,10.03 27.3,9.02 25.91,7.62 25.91,4.45 26.54,3.81 26.54,2.79 26.29,2.54 25.91,2.54 25.53,2.92 23.24,2.92 22.22,1.91 17.4,1.91 16.38,2.92 15.11,2.92 14.73,3.3 14.73,6.66 v14.94,6.86
GP77  (via drill 0.3 pad 0.64)
  Top 0.102: R23.2 11.05,25.27 11.74,25.96 11.74,27.3 10.52,28.52 v10.21,28.52
  Bottom 0.102: J1.60 5.45,27.93 5.59,28.07 5.89,28.07 6.4,27.56 8.13,27.56 8.97,28.4 10.08,28.4 v10.21,28.52
GP78  (via drill 0.1 pad 0.25 layers 1-2, 0.3 pad 0.64)
  Top 0.102: U10.14 v6.96,26.87
  Route2 0.102: v6.96,26.87 6.96,27.33 6.86,27.43 v5.79,27.43
  Bottom 0.102: J1.58 5.69,27.53 v5.79,27.43
GP79  (via drill 0.3 pad 0.64)
  Top 0.102: v6.45,28.3 7.37,27.38 U10.9
  Bottom 0.102: J1.62 6.42,28.33 v6.45,28.3
GP80  (via drill 0.3 pad 0.64)
  Top 0.102: U10.13 6.97,27.4 6.73,27.64 6.33,27.64 5.84,28.12 5.84,28.98 v6.25,29.39
  Bottom 0.102: J1.66 5.99,29.13 v6.25,29.39
GP81  (via drill 0.3 pad 0.64)
  Top 0.102: U10.17 6.44,27.27 6.04,26.87 5.51,26.87 5.21,27.18 5.21,28.45 5.33,28.57 5.33,30.35 v5.46,30.48
  Bottom 0.102: J1.70 5.29,29.93 5.46,30.1 v5.46,30.48
GP82  (via drill 0.3 pad 0.64)
  Top 0.102: U10.1 8.22,27.27 8.89,27.94 8.89,29.72 v9.02,29.84
  Bottom 0.102: J1.64 5.46,28.73 5.56,28.83 6.73,28.83 6.86,28.96 7.9,28.96 8.79,29.84 v9.02,29.84
GP83  (via drill 0.3 pad 0.64)
  Top 0.102: U10.5 7.77,27.45 8.13,27.81 8.38,27.81 8.64,28.07 8.64,29.46 8.33,29.77 v7.95,29.77
  Bottom 0.102: J1.68 5.65,29.53 6.3,30.18 7.54,30.18 v7.95,29.77
GP84  (via drill 0.1 pad 0.25 layers 1-2, 0.3 pad 0.64)
  Top 0.102: U10.18 v6.56,26.87 v6.55,26.87
  Route2 0.102: v6.55,26.87 5.51,26.87 5.08,27.3 5.08,28.07 5.84,28.83 8.51,28.83 8.89,28.45 8.89,27.94 8.51,27.56 8.51,26.92 9.65,25.78 9.65,24.05 v8.74,23.14
  Bottom 0.102: v8.74,23.14 7.15,24.73 J1.44
GP109  (via drill 0.1 pad 0.25 layers 1-2, 0.3 pad 0.64)
  Top 0.102: U12.6 11.56,17.53 11.18,17.91 11.18,18.67 10.92,18.92 v8.7,18.92 | U2.17 13.35,26.17 v13.34,26.16
  Route2 0.102: v13.34,26.16 13.34,26.42 13.08,26.67 12.75,26.67 11.84,27.58 11.84,30.96 10.92,31.88 10.92,32.13 9.91,33.15 9.65,33.15 9.02,33.78 6.98,33.78 6.35,33.15 6.35,32 5.84,31.5 5.21,31.5 4.57,30.86 4.57,29.97 3.94,29.34 3.94,27.15 v3.66,26.87 3,26.87 2.54,26.42 2.54,22.73 2.03,22.23 2.03,19.43 2.41,19.05 4.19,19.05 4.83,19.68 8.06,19.68 8.7,19.05 v8.7,18.92
  Bottom 0.102: v3.66,26.87 3.23,26.87 2.97,27.13 J1.55
GP109CH  (via drill 0.3 pad 0.64)
  Top 0.102: U11.5 16.76,6.99 v16.76,6.93 | U4.15 25.02,12.25 24.56,12.7 v24,12.7 23.75,12.95 R22.1
  Bottom 0.102: v16.76,6.93 16.76,6.6 18.29,5.08 19.3,5.08 21.34,7.11 21.34,7.87 22.8,9.34 22.8,10.35 23.75,11.3 23.75,12.45 v24,12.7
GP110  (via drill 0.1 pad 0.25 layers 1-2, 0.3 pad 0.64)
  Top 0.102: U2.16 13.15,26.67 v12.74,26.26
  Route2 0.102: v12.74,26.26 11.74,27.27 11.74,27.3 11.56,27.48 11.56,30.86 10.67,31.75 10.67,32 9.78,32.89 8.26,32.89 8,32.64 6.86,32.64 6.6,32.38 6.6,31.88 5.97,31.24 5.33,31.24 4.83,30.73 4.83,29.84 4.19,29.21 4.19,26.54 3.68,26.04 v3.43,26.04
  Bottom 0.102: J1.53 2.86,26.73 3.43,26.16 v3.43,26.04
GP111  (via drill 0.3 pad 0.64)
  Top 0.102: U16.6 8.77,33.41 8,32.64 8,30.84 v8.08,30.76 8.12,30.72 U13.1
  Route2 0.102: v8.08,30.76 8.03,30.76 7.44,30.18 5.92,30.18 5.59,29.84 5.21,29.84 4.44,29.08 4.44,26.42 4.19,26.16 4.19,25.83 v3.56,25.2
  Bottom 0.102: J1.51 2.75,26.33 2.9,26.19 2.9,25.55 3.25,25.2 v3.56,25.2
GP111CH  (via drill 0.3 pad 0.64)
  Top 0.102: v20.34,7.34 19.81,7.87 U6.5 | R19.1 v26.8,12.76 26.8,11.06 U4.12
  Bottom 0.102: v20.34,7.34 20.34,7.64 22.22,9.53 22.22,12.83 23.19,13.79 25.77,13.79 v26.8,12.76
GP114  (via drill 0.1 pad 0.25 layers 1-2, 0.3 pad 0.64)
  Top 0.102: U2.19 14.45,24.92 14.35,25.02 13.34,25.02 12.32,26.04 v12.19,26.04 | v5.51,32.28 5.78,32.02 U13.4 7.25,32.02 v7.49,32.26
  Route2 0.102: v12.19,26.04 11.81,26.04 11.56,25.78 10.92,25.78 10.67,26.04 10.67,27.33 11.3,27.96 11.3,30.73 10.41,31.62 10.41,31.88 9.65,32.64 8.51,32.64 8.13,32.26 v7.49,32.26 | v5.51,32.28 5.23,32.28 4.06,31.11 4.06,30.23 3.11,29.27 v3.11,28.38
  Bottom 0.102: J1.59 2.78,27.93 3.11,28.26 v3.11,28.38
GP114CH  (via drill 0.3 pad 0.64)
  Top 0.102: R21.1 24.83,13.53 25.15,13.21 v25.15,12.88 25.15,12.76 25.52,12.39 U4.14 | U5.5 19.94,11.3 20.32,11.68 20.32,12.37 21.29,13.34 22.05,13.34 v22.81,12.57
  Bottom 0.102: v25.15,12.88 24.51,13.51 23.29,13.51 22.81,13.03 v22.81,12.57
GP115  (via drill 0.1 pad 0.25 layers 1-2, 0.3 pad 0.64)
  Top 0.102: U2.18 13.61,25.67 v13.59,25.65 | U14.6 12.2,20.32 11.99,20.12 v10.92,20.12
  Route2 0.102: v10.92,20.12 10.54,20.5 10.54,21.34 12.83,23.62 12.83,24.89 v13.59,25.65 13.72,25.78 13.72,26.54 12.83,27.43 12.83,28.57 12.45,28.96 12.45,30.73 11.18,32 11.18,32.26 10.03,33.4 9.78,33.4 9.14,34.04 6.86,34.04 6.1,33.27 6.1,32.13 5.71,31.75 5.08,31.75 4.32,30.99 4.32,30.1 3.68,29.46 3.68,27.99 v3.3,27.61
  Bottom 0.102: J1.57 3.22,27.53 v3.3,27.61
GP115CH  (via drill 0.3 pad 0.64)
  Top 0.102: U3.5 17.91,7.87 18.62,7.16 v18.62,6.86 | U4.13 26.02,12.66 v25.97,12.7 25.78,12.89 R20.1
  Bottom 0.102: v18.62,6.86 18.29,6.53 18.29,5.59 18.54,5.33 19.18,5.33 21.08,7.24 21.08,8 22.48,9.4 22.48,10.41 23.37,11.3 23.37,12.95 23.65,13.23 24.36,13.23 24.59,13.01 24.59,12.62 24.89,12.32 25.59,12.32 v25.97,12.7
GP128  (via drill 0.1 pad 0.25 layers 1-2, 0.3 pad 0.64)
  Top 0.102: U26.3 5.6,10.8 v5.59,10.79 | v2.79,30.58 0.71,28.5 0.71,25.2 2.29,23.62 2.29,16.51 2.67,16.13 v2.67,15.49
  Route2 0.102: v2.67,15.49 2.67,13.34 5.21,10.79 v5.59,10.79
  Bottom 0.102: J1.65 2.71,29.13 2.92,29.34 2.92,30.45 v2.79,30.58
GP128CH  (via drill 0.1 pad 0.25 layers 1-2, 0.3 pad 0.64)
  Top 0.102: U26.5 7.62,10.41 v7.62,9.72 | 24.51,7.24 24.52,7.24 | 24.52,7.24 26.21,5.54 26.21,4.06 25.4,3.25 R53.2 24.83,2.35 24.59,2.11 v24.59,0.89 | U4.3 24.52,7.24
  Route2 0.102: v7.62,9.72 7.68,9.65 8.13,9.65 8.38,9.4 8.38,8.51 9.27,7.62 9.27,1.52 10.16,0.64 24.33,0.64 v24.59,0.89
GP129  (via drill 0.1 pad 0.25 layers 1-2, 0.3 pad 0.64)
  Top 0.102: U27.3 7.49,8.51 6.6,9.4 6.6,9.78 6.1,10.29 5.21,10.29 v4.95,10.54 | v1.52,30.5 0.46,29.44 0.46,25.07 2.03,23.5 2.03,16.76 v1.78,16.51
  Route2 0.102: v4.95,10.54 4.95,10.67 1.52,14.1 1.52,16.26 v1.78,16.51
  Bottom 0.102: J1.63 1.32,28.73 1.22,28.83 1.22,30.2 v1.52,30.5
GP129CH  (via drill 0.1 pad 0.25 layers 1-2, 0.3 pad 0.64)
  Top 0.102: U4.5 25.52,7 26.54,5.97 26.92,5.97 | U27.5 8.89,9.02 v9.27,8.64 | R48.2 28.19,7.37 27.3,6.48 27.3,6.35 27.05,6.1 | 27.05,5.97 26.92,5.97 | 27.05,5.84 27.05,5.97 | 27.05,5.97 27.05,6.1 | 26.92,5.97 27.05,6.1 | 26.92,5.97 27.05,5.84 | 27.05,5.84 27.05,5.17 v27.08,5.14
  Route2 0.102: v9.27,8.64 9.4,8.51 9.4,8.26 9.78,7.87 9.78,1.91 10.54,1.14 23.43,1.14 24.19,1.91 26.54,1.91 27.81,3.17 27.81,4.7 27.37,5.14 v27.08,5.14
GP130  (via drill 0.1 pad 0.25 layers 1-2, 0.3 pad 0.64)
  Top 0.102: U9.3 v14.1,10.79
  Route2 0.102: v14.1,10.79 14.22,10.92 14.22,11.68 13.72,12.19 13.72,13.84 13.59,13.97 13.59,18.8 13.08,19.3 13.08,21.84 13.59,22.35 13.84,22.35 14.22,22.73 14.22,23.24 13.97,23.5 13.97,24.77 14.48,25.27 14.48,28.7 15.11,29.34 15.11,30.23 14.73,30.61 13.84,30.61 13.08,31.37 13.08,34.16 11.43,35.81 9.4,35.81 8.38,34.8 6.48,34.8 2.97,31.29 v1.35,31.29
  Bottom 0.102: J1.61 1.21,28.33 0.96,28.57 0.96,30.91 v1.35,31.29
GP130CH  (via drill 0.1 pad 0.25 layers 1-2, 0.3 pad 0.64)
  Top 0.102: U4.1 23.52,7.51 23.11,7.11 22.48,7.11 21.21,5.84 v21.21,2.41 21.27,2.35 R16.2 | U9.5 14.99,11.3 15.24,11.05 15.24,10.54 15.56,10.22 v15.74,10.22
  Route2 0.102: v15.74,10.22 15.74,9.51 15.37,9.14 15.37,8.64 15.75,8.26 15.75,3.94 17.4,2.29 21.08,2.29 v21.21,2.41
GP131  (via drill 0.1 pad 0.25 layers 1-2, 0.3 pad 0.64)
  Top 0.102: U8.3 12.25,10.8 v12.26,10.79
  Route2 0.102: v12.26,10.79 12.45,10.99 12.45,11.81 12.07,12.19 12.07,16.32 11.05,17.34 11.05,18.99 9.97,20.07 9.97,21.91 v11.25,23.19
  Bottom 0.102: J1.46 5.57,25.13 5.97,25.53 6.73,25.53 7.24,25.02 7.87,25.02 10.03,22.86 10.92,22.86 v11.25,23.19
GP131CH  (via drill 0.1 pad 0.25 layers 1-2, 0.3 pad 0.64)
  Top 0.102: U8.5 12.83,11.3 13.34,10.79 13.34,10.49 v13.41,10.41 | U4.2 24.02,7.35 25.91,5.46 25.91,4.19 24.08,2.36 v23.47,2.36 23.46,2.35 R17.2
  Route2 0.102: v13.41,10.41 13.08,10.08 13.08,9.27 12.38,8.57 12.38,7.81 12.19,7.62 12.19,2.79 13.34,1.65 22.76,1.65 v23.47,2.36
GP134  (via drill 0.3 pad 0.64)
  Top 0.102: J9.7 27.3,19.93 28.32,20.95 v29.08,20.95
  Bottom 0.102: J1.22 5.47,20.33 5.59,20.45 5.59,21.97 6.6,22.99 7.75,22.99 8.38,22.35 13.84,22.35 14.73,23.24 18.67,23.24 19.3,23.88 27.56,23.88 28.83,22.61 28.83,21.21 v29.08,20.95
GP135  (via drill 0.3 pad 0.64)
  Top 0.102: J9.6 27.63,19.43 v28.51,20.32
  Route2 0.102: v7.49,22.38 6.71,21.59 5.97,21.59 5.71,21.84 4.06,21.84 3.68,21.46 v3.3,21.46
  Bottom 0.102: J1.27 3.24,21.53 v3.3,21.46 | v7.49,22.38 7.49,22.35 7.75,22.1 13.97,22.1 14.83,22.96 18.77,22.96 19.43,23.62 27.43,23.62 28.51,22.54 v28.51,20.32
GP183  (via drill 0.3 pad 0.64)
  Top 0.102: U7.3 11.2,8.15 v10.83,8.15 10.5,8.15 R30.1
  Route2 0.102: v10.83,8.15 10.83,8.22 10.41,8.64 10.41,9.78 11.18,10.54 11.18,11.43 10.92,11.68 10.67,11.68 10.29,12.06 10.29,16.38 10.03,16.64 10.03,18.49 8.08,20.45 2.79,20.45 2.29,20.95 2.29,22.1 2.92,22.73 v3.17,22.73
  Bottom 0.102: J1.39 2.74,23.93 2.9,23.77 2.9,23.01 v3.17,22.73
GP183CH  (via drill 0.3 pad 0.64)
  Top 0.102: U7.5 12.24,8.89 12.4,8.74 12.4,7.32 v12.8,6.91 | U4.11 27.36,10.53 27.62,10.79 v27.62,11.43 R52.1 28.26,11.68
  Bottom 0.102: v12.8,6.91 12.8,5.99 14.73,4.06 14.73,3.43 14.99,3.17 15.62,3.17 17.02,4.57 19.3,4.57 21.97,7.24 25.4,7.24 26.29,8.13 27.56,8.13 28.07,8.64 28.07,10.99 v27.62,11.43
N$1
  Top 0.305: R27.1 19.94,21.53 R1.2
N$2
  Top 0.254: SYS.+ 29.46,26.35 R70.2
N$3
  Bottom 0.102: J1.31 0.97,22.33 PCVR.T
N$4
  Top 0.102: U28.6 21.85,17.78 22.03,17.59 R24.2 21.21,17.02 | 21.21,17.02 21.14,17.02 R25.1 21.02,16.95 21.21,17.14 21.14,17.14 21.08,17.14 | 21.08,17.14 21.21,17.02 | 21.21,17.02 21.21,16.89 21.08,16.76 21.08,17.14
N$5
  Top 0.254: R31.2 CHR.+
N$6  (via drill 0.1 pad 0.25 layers 1-2, 0.3 pad 0.64)
  Top 0.102: U11.3 | U12.1 10.68,18.53 10.92,18.29 10.92,17.78 12.07,16.64 14.29,16.64 v14.35,16.7
  Route2 0.102: U11.3 15.49,7.49 15.49,8.13 15.11,8.51 15.11,9.4 15.37,9.65 15.37,11.3 15.88,11.81 15.88,14.5 v16.4,15.02
  Bottom 0.102: v16.4,15.02 16.4,15.48 16,15.88 15.18,15.88 v14.35,16.7
  other vias: 15.37,7.37
N$7
  Top 0.254: CHR.- 28.45,30.1 U19.9
N$8
  Top 0.305: U2.1 20.17,25.67 L1.2
N$9
  Top 0.102: U2.5 19.89,27.67 R4.1
N$10
  Top 0.102: U2.3 19.05,26.67 19.18,26.8 19.18,27.05 19.05,27.17 U2.4
N$11
  Top 0.305: U28.2 22.35,20.23 22.35,20.44 | 22.35,20.44 22.35,20.45 | 22.35,20.44 22.35,21.08
  pour Top (isolate 0.254, no thermals): 22.22,19.66 22.22,20.7 21.95,20.98 21.95,22.3 22.02,22.38 23.24,22.38 23.34,22.28 23.34,21.55 22.48,20.69 22.48,19.68 22.43,19.63 22.25,19.63
N$12
  Top 0.102: U2.23 R5.1
N$13
  Top 0.102: U4.23 22.11,9.03 21.84,8.76 21.84,8.13 21.65,7.94 R44.1
N$14
  Top 0.102: U2.24 17.51,23.83 R6.1 R7.1
N$15
  Top 0.102: U2.13 13.14,28.17 C8.2 R8.1
N$16
  Top 0.102: U2.9 16.51,29.85 16.26,30.1 C12.2 15.72,31.33 15.72,32.23 15.81,32.32 R12.1
N$17
  Top 0.102: U2.8 17.01,30.09 17.27,30.35 C13.2 R13.1
N$18
  Top 0.102: R9.1 C9.2 12.76,30.8 13.84,29.72 13.84,29.46 14.38,28.92 U2.12
N$19
  Top 0.102: U2.11 15.51,29.45 14.61,30.35 14.35,30.35 13.91,30.8 C10.2 13.4,30.8 13.27,30.92 13.27,32.38 R10.1
N$20
  Top 0.102: U2.10 16.01,29.4 14.99,30.42 C11.2 14.54,30.8 14.41,30.92 14.41,32.64 R11.1
N$21  (via drill 0.3 pad 0.64)
  Top 0.102: J2.15 3.91,17.75 3.43,17.27 3.43,12.02 2.08,10.67 v1.52,10.67
  Bottom 0.102: P1.MM v1.52,10.67
N$23  (via drill 0.1 pad 0.25 layers 1-2)
  Top 0.102: U3.3 v17.27,7.37 | U14.1 10.41,21.32 10.78,21.69 13.74,21.69 v14.22,21.21
  Route2 0.102: v17.27,7.37 17.27,7.95 16.64,8.59 16.64,9.78 16.13,10.29 16.13,11.68 16.7,12.26 16.76,12.32 16.89,12.45 16.89,15.62 14.61,17.91 14.61,19.43 14.22,19.81 v14.22,21.21
N$24  (via drill 0.3 pad 0.64)
  Top 0.102: J2.16 4.04,17.25 3.68,16.89 3.68,13.27 v4,12.95
  Bottom 0.102: P2.MM 4.7,10.67 4.95,10.92 4.95,12.7 4.7,12.95 v4,12.95
N$27
  Top 0.102: U18.1 4.22,7.46 2.79,8.89 R59.2
N$28
  Top 0.102: U18.10 6.47,2.92 6.35,2.79 5.84,2.79 5.54,2.49 4.8,2.49 4.63,2.32 R58.1
N$29
  Top 0.102: U18.15 8.77,5.21 8.89,5.33 8.89,6.54 R54.1
N$30
  Top 0.102: U18.12 7.47,1.99 R57.1
N$31
  Top 0.102: U18.13 9.29,4.21 9.71,4.64 R56.1
N$32
  Top 0.102: U18.14 8.9,4.71 9.14,4.95 9.14,5.78 R55.1
N$33
  Top 0.102: U18.2 3.7,6.21 3.56,6.35 3.56,7.75 3.3,8 R60.2
N$34
  Top 0.102: U18.8 5.47,2.98 5.28,2.79 4.83,2.79 4.57,3.05 4.57,3.3 4.32,3.56 R61.2
N$35
  Top 0.102: U10.19 6.4,26.47 6.35,26.42 5.33,26.42 4.74,27.01 R14.1
N$36
  Top 0.102: U18.11 6.97,2.78 6.68,2.49 6.24,2.49 R64.1
N$37
  Top 0.102: U18.5 3.42,4.71 2.79,5.33 R62.2
N$38
  Top 0.102: R63.2 3.3,6.54 3.3,6.1 3.69,5.71 U18.3
N$39
  Top 0.102: U18.4 3.81,5.21 2.79,6.22 R65.2
N$40
  Top 0.102: U18.6 2.96,4.21 R66.2
N$43
  Top 0.102: U4.18 23.52,12.43 23.37,12.57 23.37,12.95 22.8,13.53 R45.1
N$44  (via drill 0.1 pad 0.25 layers 1-2, 0.3 pad 0.64)
  Top 0.102: U5.3 v19.18,10.79 | U15.1 10.68,24.25 v10.79,24.13
  Route2 0.102: v19.18,10.79 19.18,11.05 20.32,12.19 20.32,12.7 19.81,13.21 19.81,16.89 20.45,17.53 20.45,19.3 18.41,21.34 18.41,23.37 18.03,23.75 v18.03,24.13
  Bottom 0.102: v10.79,24.13 11.18,24.13 11.81,23.5 17.4,23.5 v18.03,24.13
N$45
  Top 0.254: 21.02,22.73 21.02,22.86 R26.2
  Top 0.305: U28.4 21.35,21.39 R1.1 21.02,22.73
N$46  (via drill 0.3 pad 0.64)
  Top 0.102: R35.1 28.96,35.81 28.57,36.2 26.42,36.2 v26.16,35.94
  Bottom 0.102: FW_RCVR.2 26.27,35.84 v26.16,35.94
N$47
  pour Top (isolate 0.254, no thermals): 25.53,30.73 24.89,30.73 24.77,30.61 24.77,29.72 24.51,29.46 23.49,29.46 23.37,29.34 23.37,27.94 23.62,27.69 25.4,27.69 25.65,27.94 25.65,30.61
N$48  (via drill 0.1 pad 0.25 layers 1-2, 0.3 pad 0.64)
  Top 0.102: U6.3 | U16.1 7.25,34.41 7.57,34.09 v7.57,33.27
  Route2 0.102: U6.3 19.18,8.33 19,8.51 19,9.09 19.3,9.4 19.3,10.16 19.56,10.41 19.56,11.05 20.57,12.06 20.57,12.83 20.07,13.34 20.07,16.76 20.7,17.4 20.7,19.43 18.67,21.46 18.67,27.81 17.65,28.83 v17.65,30
  Bottom 0.102: v7.57,33.27 9.53,33.27 11.68,31.11 16.54,31.11 v17.65,30
  other vias: 19.18,7.37
N$50
  Top 0.203: R38.2 3V3.+
N$51
  Top 0.203: 1V8.+ R39.2
N$53  (via drill 0.3 pad 0.64)
  Top 0.102: v28.57,32.51 28.7,32.51 28.96,32.26 28.96,31.88 28.69,31.61 U19.12 | v25.78,28.45 25.78,28.26 R28.1
  Bottom 0.102: v28.57,32.51 28.19,32.13 28.19,30.73 25.91,28.45 v25.78,28.45
N$58  (via drill 0.3 pad 0.64)
  Top 0.102: U19.11 28.9,31.11 v29.08,30.92 | v26.67,28.45 26.67,28.13 R29.1
  Bottom 0.102: v26.67,28.45 26.67,28.51 v29.08,30.92
N$76  (via drill 0.3 pad 0.64)
  Top 0.102: R34.1 R32.2 v28.7,12.51
  Bottom 0.102: PWR.2 27.28,9.29 26.92,9.65 26.92,11.87 27.56,12.51 v28.7,12.51
N$78  (via drill 0.1 pad 0.25 layers 1-2)
  Top 0.102: U15.6 12.2,23.25 11.94,22.99 11.94,22.61 11.46,22.12 9.75,22.12 v9.65,22.23 | U13.2 9.4,31.37 10.41,30.35 v10.57,30.35
  Route2 0.102: v9.65,22.23 9.65,23.62 10.16,24.13 10.16,27.61 10.79,28.25 10.79,30.12 v10.57,30.35
PSW  (via drill 0.3 pad 0.64)
  Top 0.102: 26.19,17.5 26.29,17.4 26.32,17.43 | v0.76,20.83 v0.76,17.78 | J9.2 26.32,17.43 | 26.32,17.43 26.51,17.43 26.67,17.27 26.67,16.4 v25.59,15.32
  Bottom 0.102: J1.21 1.26,20.33 v0.76,20.83 | v0.76,17.78 0.76,16.38 2.03,15.11 4.95,15.11 5.33,14.73 5.33,14.22 6.1,13.46 11.05,13.46 11.3,13.72 22.73,13.72 23.11,14.1 25.02,14.1 25.59,14.67 v25.59,15.32
PWM0  (via drill 0.1 pad 0.25 layers 1-2, 0.3 pad 0.64)
  Top 0.102: U22.4 v17.78,10.79 | J2.13 4.27,18.75 4.14,18.62 4.14,18.5 v3.94,18.29 3.17,17.53 3.17,12.15 2.32,11.3 1.4,11.3 0.89,10.79 0.89,6.6 1.27,6.22 R65.1
  Route2 0.102: v3.94,18.29 4.27,18.62 7.62,18.62 7.82,18.41 8.64,18.41 9.33,17.72 v9.33,16.04 | v17.78,10.79 17.27,11.3 17.27,14.95 v17.91,15.58
  Bottom 0.102: v9.33,16.04 9.55,16.26 12.95,16.26 13.97,17.27 14.54,17.27 15.68,16.13 17.36,16.13 v17.91,15.58
PWM0CH  (via drill 0.1 pad 0.25 layers 1-2, 0.3 pad 0.64)
  Top 0.102: U22.5 18.16,10.92 18.16,10.41 17.96,10.21 v17.47,10.21 | R51.2 26.36,2.4 26.36,2.81 v26.05,3.12 26.54,3.62 26.54,5.59 25.02,7.12 U4.4
  Route2 0.102: v17.47,10.21 17.32,10.21 16.89,9.78 16.89,8.71 17.65,7.95 17.65,7.24 17.4,6.99 17.4,6.73 17.14,6.48 16.38,6.48 16.13,6.22 16.13,4.57 16,4.45 16,4.06 17.53,2.54 20.57,2.54 20.99,2.95 21.16,3.12 21.27,3.24 25.97,3.24 26.05,3.16 v26.05,3.12
PWM1  (via drill 0.1 pad 0.25 layers 1-2, 0.3 pad 0.64)
  Top 0.102: U23.4 v8.76,10.79 | J2.14 5.93,18.25 v5.94,18.26 | R66.1 v1.14,4.45
  Route2 0.102: v5.94,18.26 6.04,18.36 7.42,18.36 8.13,17.65 8.13,16.51 9.08,15.56 9.46,15.56 9.78,15.24 9.78,14.48 9.02,13.72 8.64,13.72 8.13,13.21 8.13,12.06 8.76,11.43 v8.76,10.79 8.13,10.79 7.24,9.91 7.24,8.76 7.49,8.51 8,8.51 9.02,7.49 9.02,5.38 7.57,3.94 1.65,3.94 v1.14,4.45
PWM1CH  (via drill 0.1 pad 0.25 layers 1-2, 0.3 pad 0.64)
  Top 0.102: U4.6 26.02,7.26 v26.73,6.54 27.37,7.18 27.37,7.56 28.19,8.38 R50.2 | v9.22,10.79 9.22,10.85 U23.5
  Route2 0.102: v9.22,10.79 9.22,10.36 8.64,9.78 8.64,8.64 9.53,7.75 9.53,1.78 10.41,0.89 23.62,0.89 24.38,1.65 26.67,1.65 28.07,3.05 28.07,5.21 v26.73,6.54
PWM3  (via drill 0.1 pad 0.25 layers 1-2, 0.3 pad 0.64)
  Top 0.102: v8.23,3.3 8.87,3.94 11.1,3.94 11.56,4.39 11.56,5.84 11.81,6.1 11.81,7.62 11.68,7.75 v11.68,8 11.93,8.25 U7.4 | R64.2 6.6,1.91 v6.6,1.21 | J2.8 5.27,21.25 v5.28,21.23 5.32,21.2
  Route2 0.102: v8.23,3.3 8.23,2.83 v6.6,1.21 | v11.68,8 11.68,10.73 12.19,11.24 12.19,11.68 11.81,12.06 11.81,15.37 11.3,15.88 11.3,16.26 10.54,17.02 10.54,18.75 8.31,20.98 5.54,20.98 v5.28,21.23
PWRBTN_N  (via drill 0.3 pad 0.64)
  Top 0.102: R34.2 28.7,13.4 v28.69,13.41
  Bottom 0.102: J1.17 2.95,19.53 3.68,18.8 3.68,15.88 3.94,15.62 5.84,15.62 7.49,13.97 10.79,13.97 11.05,14.22 22.44,14.22 22.85,14.63 24.15,14.63 24.51,14.99 24.51,15.75 24.89,16.13 27.18,16.13 PWRBT.T 28.7,13.42 v28.69,13.41
SCL  (via drill 0.3 pad 0.64)
  Top 0.102: U18.19 7.47,8.15 v5.97,9.65 | v9.02,14.8 9.02,14.73 9.53,14.22 Q2.3 9.53,14.1 R43.1 | U4.19 22.77,11.44 v22.83,11.51
  Route2 0.102: v5.97,9.65 6.22,9.65 7.11,10.54 7.11,11.81 7.49,12.19 7.49,13.46 8.26,14.22 8.76,14.22 9.02,14.48 v9.02,14.8 9.02,14.86 | v22.83,11.51 22.86,11.48 22.86,9.4 21.34,7.87 21.34,3.68 20.68,3.02 v17.91,3.02
  Bottom 0.102: v5.97,9.65 5.97,9.02 5.51,8.56 5.51,8 5.77,7.75 6.98,7.75 10.6,4.13 13.08,4.13 13.65,3.56 13.65,1.84 14.1,1.4 17.02,1.4 17.91,2.29 v17.91,3.02 17.91,3.94 18.16,4.19 18.92,4.19 19.18,3.94 21.08,3.94 23.24,1.78 25.4,1.78 SCL.T
SCL6  (via drill 0.1 pad 0.25 layers 1-2, 0.3 pad 0.64)
  Top 0.102: R67.1 3.68,39.05 Q4.3 v4.95,38.48 | J4.9 13.88,36.76 v14.1,36.98 | J3.4 13.88,5.88 v13.91,5.91
  Route2 0.102: v14.1,36.98 14.1,34.67 14.61,34.16 14.61,31.88 15.88,30.61 15.88,28.96 15.24,28.32 15.24,24.89 14.8,24.45 14.8,23.8 14.99,23.62 14.99,22.35 14.22,21.59 13.97,21.59 13.84,21.46 13.84,19.68 14.35,19.18 14.35,17.78 15.11,17.02 15.11,15.11 15.49,14.73 15.49,11.94 14.99,11.43 14.99,9.91 14.86,9.78 14.86,8.51 14.48,8.13 14.48,6.99 14.35,6.86 14.35,6.35 v13.91,5.91
  Bottom 0.102: v14.1,36.98 14.07,36.98 12.57,38.48 SCL6.T v4.95,38.48
SDA  (via drill 0.3 pad 0.64)
  Top 0.102: U18.20 6.97,8.27 6.22,9.02 v5.21,9.02 | U4.20 22.24,10.53 22.1,10.67 22.1,12.34 v21.67,12.78 | R41.1 15.18,13.91 Q1.3 15.49,15.23 v15.62,15.35
  Route2 0.102: v18.52,3.63 20.52,3.63 21.08,4.19 21.08,8.26 22.1,9.27 22.1,12.34 v21.67,12.78 21.46,12.98 21.46,14.55 v21.26,14.76
  Bottom 0.102: v5.21,9.02 5.21,7.87 5.59,7.49 6.86,7.49 10.48,3.87 12.83,3.87 13.4,3.3 13.4,1.71 13.97,1.14 17.65,1.14 18.52,2.01 v18.52,3.63 21.01,3.63 23.11,1.52 SDA.T | v15.62,15.35 15.62,14.73 15.88,14.48 20.98,14.48 v21.26,14.76
SDA6  (via drill 0.1 pad 0.25 layers 1-2, 0.3 pad 0.64)
  Top 0.102: R3.1 4.19,36.13 Q3.3 5.08,37.02 v5.08,37.24 | J4.10 13.38,36.69 v13.34,36.73 | J3.3 13.38,4.02 v13.46,3.94
  Route2 0.102: v13.34,36.73 13.34,36.2 13.59,35.94 13.59,34.8 14.35,34.04 14.35,31.75 15.62,30.48 15.62,29.08 14.99,28.45 14.99,25.02 14.55,24.58 14.55,23.68 14.73,23.5 14.73,22.48 14.1,21.84 13.84,21.84 13.59,21.59 13.59,19.56 14.1,19.05 14.1,17.65 14.86,16.89 14.86,14.99 15.24,14.61 15.24,12.06 14.73,11.56 14.73,10.03 14.61,9.91 14.61,8.64 14.15,8.18 14.15,7.04 13.46,6.35 v13.46,3.94
  Bottom 0.102: v13.34,36.73 12.83,37.24 v5.08,37.24 5.1,37.21 SDA6.T
SPI_CLK/D13  (via drill 0.1 pad 0.25 layers 1-2, 0.3 pad 0.64)
  Top 0.102: R54.2 v11.28,7.37 | J4.1 17.88,36.67 v17.91,36.7 | v17.86,5.56 17.88,5.54 J3.12 17.88,4.16 16.23,2.52 v16.23,2.39 | U11.4 15.87,6.89 v16.64,6.12
  Route2 0.102: v17.91,36.7 17.91,31.88 16.89,30.86 16.89,28.83 18.16,27.56 18.16,25.65 17.27,24.77 17.27,23.75 17.91,23.11 17.91,21.08 19.94,19.05 19.94,17.78 19.3,17.14 19.3,13.08 17.91,11.68 17.91,11.18 18.16,10.92 18.16,10.29 17.14,9.27 17.14,8.84 17.91,8.08 17.91,7.11 17.65,6.86 17.65,6.6 17.17,6.12 v16.64,6.12 16.64,5.84 16.92,5.56 v17.86,5.56
  Bottom 0.102: v11.28,7.37 11.28,7.14 14.48,3.94 14.48,3.17 14.73,2.92 15.75,2.92 16.23,2.44 v16.23,2.39
SPI_CS/D10  (via drill 0.1 pad 0.25 layers 1-2, 0.3 pad 0.64)
  Top 0.102: U6.4 v19.68,6.74 v19.68,6.73 v19.68,4.19 19.68,3.94 16.64,0.89 8.89,0.89 8.45,1.33 R57.2 | J3.9 v16.38,4.2 v16.38,4.19 | J4.4 16.38,35.95 v16,36.32
  Route2 0.102: v16.38,4.19 v19.68,4.19 | v16,36.32 16,37.21 16.51,37.72 18.41,37.72 18.92,37.21 18.92,35.81 18.67,35.56 18.67,31.5 18.41,31.24 18.41,28.83 19.18,28.07 19.18,21.72 21.21,19.68 21.21,19.05 21.97,18.29 21.97,17.14 20.57,15.75 20.57,13.59 21.08,13.08 21.08,12.29 v21.37,12
  Bottom 0.102: v19.68,6.73 19.68,7.75 20.42,8.48 20.42,11.02 21.37,11.98 v21.37,12
SPI_MISO/D12  (via drill 0.1 pad 0.25 layers 1-2, 0.3 pad 0.64)
  Top 0.102: R55.2 v11.25,6.35 | U5.4 19.68,10.03 v19.81,9.91 | v16.89,5.08 16.88,5.07 J3.10 16.88,4.08 15.97,3.17 15.37,3.17 v14.48,2.29 | J4.3 16.88,35.83 16.57,36.13 v16.57,36.89
  Route2 0.102: v16.89,5.08 18.03,5.08 v18.92,5.97 | v16.57,36.89 17.14,37.47 18.29,37.47 18.67,37.08 18.67,35.94 18.41,35.69 18.41,31.62 18.16,31.37 18.16,28.7 18.92,27.94 18.92,21.59 20.95,19.56 20.95,18.92 21.72,18.16 21.72,17.27 20.32,15.88 20.32,13.46 20.83,12.95 20.83,11.94 19.81,10.92 v19.81,9.91
  Bottom 0.102: v18.92,5.97 19.15,6.2 19.15,7.59 20.14,8.59 20.14,9.58 v19.81,9.91 | v14.48,2.29 14.22,2.54 14.22,3.81 11.68,6.35 v11.25,6.35
SPI_MOSI/D11  (via drill 0.1 pad 0.25 layers 1-2, 0.3 pad 0.64)
  Top 0.102: U3.4 18.01,7.14 v18.01,6.58 17.38,5.95 J3.11 17.38,4.17 16.13,2.92 15.75,2.92 15.37,2.54 v15.37,2.29 | R56.2 10.6,4.89 10.79,4.7 v10.99,4.7 | J4.2 17.38,36.09 v17.14,36.32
